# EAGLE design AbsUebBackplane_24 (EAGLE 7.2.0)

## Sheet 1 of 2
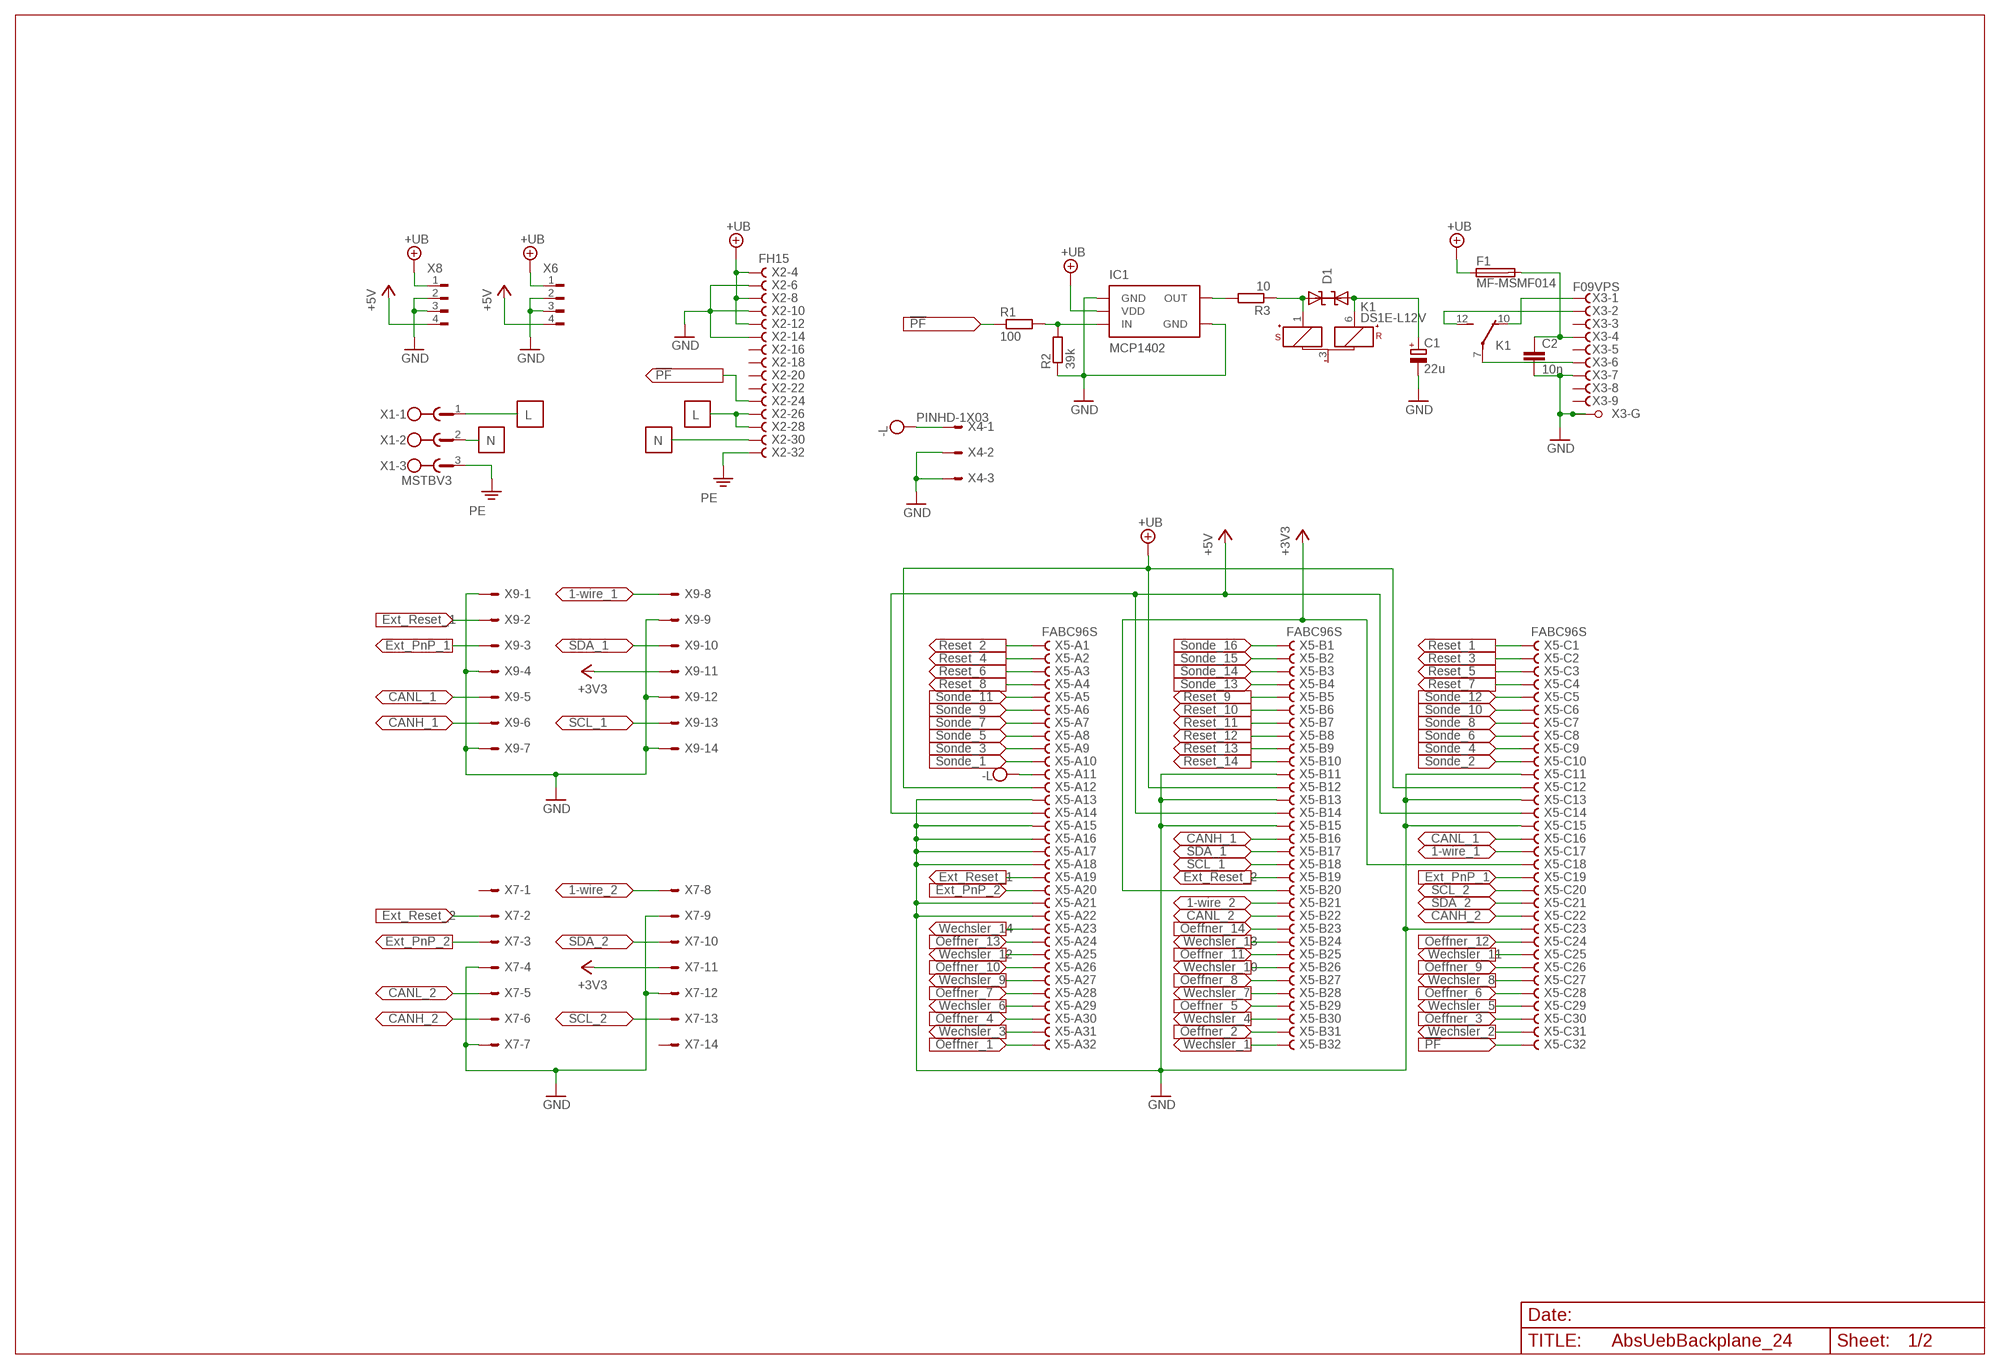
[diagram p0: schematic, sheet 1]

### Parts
C1  22u  CPOL-2-5  [RAD-FR-2,0-5]
C2  10n  C-SMD-1206  [C1206]
D1  P6SMB11CAT3  [SMB-DO-214AA]
F1  MF-MSMF014  [MF-MSMF-S1]
IC1  MCP1402  [SOT223-5]
K1  DS1E-L12V  [DS1E-L]
R1  100  R-SMD-1206  [R1206]
R2  39k  R-SMD-1206  [R1206]
R3  10  R-SMD-1206  [R1206]
X1  MSTBV3  [MSTBV3]
X2  FH15  [FH15]
X3  F09VPS  [F09VP]
X4  PINHD-1X03  [PINHD-1X03_LOCK]
X5  FABC96S  [FABC96S]
X6  FLOPPY-4  [FLOPPY-4]
X7  ML14E  [ML14]
X8  FLOPPY-4  [FLOPPY-4]
X9  ML14E  [ML14]

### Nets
1-WIRE_1: X5.C17 X9.8
1-WIRE_2: X5.B21 X7.8
!PF: R1.1 X2.24 X5.C32
+3V3: X5.B20 X5.C18 X7.11 X9.11
+5V: X5.A14 X5.B14 X5.C14 X6.4 X8.4
+UB: F1.1 IC1.2(VDD) X2.4 X2.8 X2.12 X5.A12 X5.B12 X5.C12 X6.1 X8.1 ; also sheet 2
-L: X4.1 X5.A11 ; also sheet 2
CANH_1: X5.B16 X9.6
CANH_2: X5.C22 X7.6
CANL_1: X5.C16 X9.5
CANL_2: X5.B22 X7.5
EXT_PNP_1: X5.C19 X9.3
EXT_PNP_2: X5.A20 X7.3
EXT_RESET_1: X5.A19 X9.2
EXT_RESET_2: X5.B19 X7.2
GND: C1.- C2.2 IC1.1(GND) IC1.4(GND) R2.1 X2.6 X2.10 X2.14 X3.7(-7:F) X3.G1(-G:G1) X3.G2(-G:G2) X4.2 X4.3 X5.A13 X5.A15 X5.A16 X5.A17 X5.A18 X5.A21 X5.A22 X5.B11 X5.B13 X5.B15 X5.C11 X5.C13 X5.C15 X5.C23 X6.2 X6.3 X7.4 X7.7 X7.9 X7.12 X8.2 X8.3 X9.1 X9.4 X9.7 X9.9 X9.12 X9.14 ; also sheet 2
L: X1.1 X2.26 X2.28
N: X1.2 X2.30
N$1: D1.1(C) K1.1(1:S+) R3.1
N$2: IC1.3(IN) R1.2 R2.2
N$3: C1.+ D1.2(A) K1.6(1:R+)
N$4: IC1.5(OUT) R3.2
N$5: K1.7(2:P) X3.6(-6:F)
N$6: K1.10(2:O) X3.1(-1:F)
N$7: K1.12(2:S) X3.2(-2:F)
N$8: C2.1 F1.2 X3.4(-4:F)
OEFFNER_1: X5.A32 ; also sheet 2
OEFFNER_2: X5.B31 ; also sheet 2
OEFFNER_3: X5.C30 ; also sheet 2
OEFFNER_4: X5.A30 ; also sheet 2
OEFFNER_5: X5.B29 ; also sheet 2
OEFFNER_6: X5.C28 ; also sheet 2
OEFFNER_7: X5.A28 ; also sheet 2
OEFFNER_8: X5.B27 ; also sheet 2
OEFFNER_9: X5.C26 ; also sheet 2
OEFFNER_10: X5.A26 ; also sheet 2
OEFFNER_11: X5.B25 ; also sheet 2
OEFFNER_12: X5.C24 ; also sheet 2
OEFFNER_13: X5.A24 ; also sheet 2
OEFFNER_14: X5.B23 ; also sheet 2
PE: X1.3 X2.32
RESET_1: X5.C1 ; also sheet 2
RESET_2: X5.A1 ; also sheet 2
RESET_3: X5.C2 ; also sheet 2
RESET_4: X5.A2 ; also sheet 2
RESET_5: X5.C3 ; also sheet 2
RESET_6: X5.A3 ; also sheet 2
RESET_7: X5.C4 ; also sheet 2
RESET_8: X5.A4 ; also sheet 2
RESET_9: X5.B5 ; also sheet 2
RESET_10: X5.B6 ; also sheet 2
RESET_11: X5.B7 ; also sheet 2
RESET_12: X5.B8 ; also sheet 2
RESET_13: X5.B9 ; also sheet 2
RESET_14: X5.B10 ; also sheet 2
SCL_1: X5.B18 X9.13
SCL_2: X5.C20 X7.13
SDA_1: X5.B17 X9.10
SDA_2: X5.C21 X7.10
SONDE_1: X5.A10 ; also sheet 2
SONDE_2: X5.C10 ; also sheet 2
SONDE_3: X5.A9 ; also sheet 2
SONDE_4: X5.C9 ; also sheet 2
SONDE_5: X5.A8 ; also sheet 2
SONDE_6: X5.C8 ; also sheet 2
SONDE_7: X5.A7 ; also sheet 2
SONDE_8: X5.C7 ; also sheet 2
SONDE_9: X5.A6 ; also sheet 2
SONDE_10: X5.C6 ; also sheet 2
SONDE_11: X5.A5 ; also sheet 2
SONDE_12: X5.C5 ; also sheet 2
SONDE_13: X5.B4 ; also sheet 2
SONDE_14: X5.B3 ; also sheet 2
SONDE_15: X5.B2
SONDE_16: X5.B1
WECHSLER_1: X5.B32 ; also sheet 2
WECHSLER_2: X5.C31 ; also sheet 2
WECHSLER_3: X5.A31 ; also sheet 2
WECHSLER_4: X5.B30 ; also sheet 2
WECHSLER_5: X5.C29 ; also sheet 2
WECHSLER_6: X5.A29 ; also sheet 2
WECHSLER_7: X5.B28 ; also sheet 2
WECHSLER_8: X5.C27 ; also sheet 2
WECHSLER_9: X5.A27 ; also sheet 2
WECHSLER_10: X5.B26 ; also sheet 2
WECHSLER_11: X5.C25 ; also sheet 2
WECHSLER_12: X5.A25 ; also sheet 2
WECHSLER_13: X5.B24 ; also sheet 2
WECHSLER_14: X5.A23 ; also sheet 2
Unconnected: K1.3(1:-) X2.16 X2.18 X2.20 X2.22 X3.3(-3:F) X3.5(-5:F) X3.8(-8:F) X3.9(-9:F) X7.1 X7.14

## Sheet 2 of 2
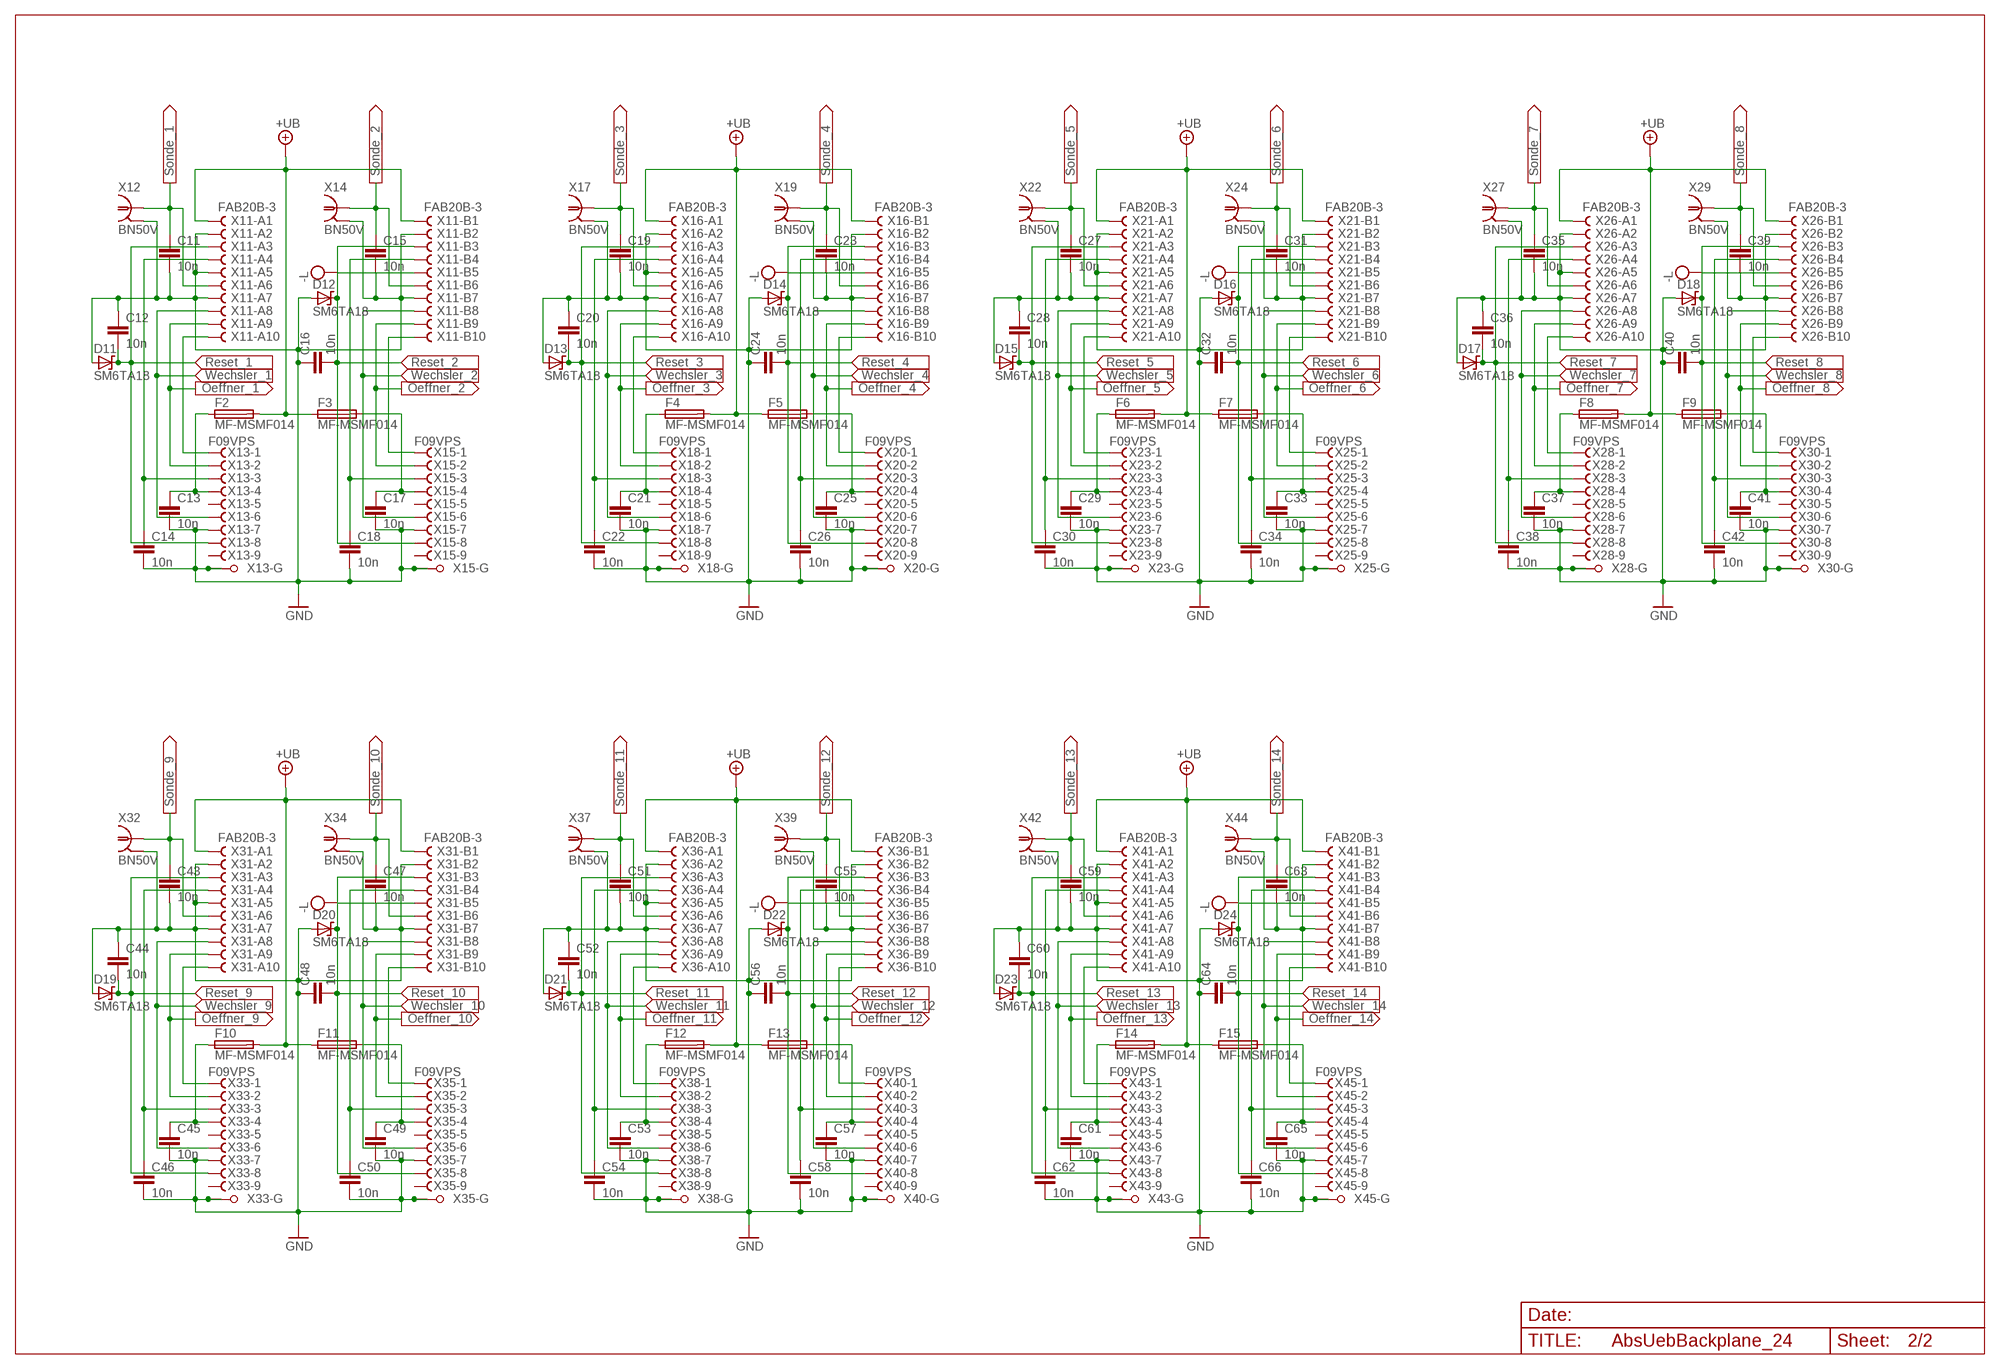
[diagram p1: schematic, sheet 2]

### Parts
C11  10n  C-SMD-1206  [C1206]
C12  10n  C-SMD-1206  [C1206]
C13  10n  C-SMD-1206  [C1206]
C14  10n  C-SMD-1206  [C1206]
C15  10n  C-SMD-1206  [C1206]
C16  10n  C-SMD-1206  [C1206]
C17  10n  C-SMD-1206  [C1206]
C18  10n  C-SMD-1206  [C1206]
C19  10n  C-SMD-1206  [C1206]
C20  10n  C-SMD-1206  [C1206]
C21  10n  C-SMD-1206  [C1206]
C22  10n  C-SMD-1206  [C1206]
C23  10n  C-SMD-1206  [C1206]
C24  10n  C-SMD-1206  [C1206]
C25  10n  C-SMD-1206  [C1206]
C26  10n  C-SMD-1206  [C1206]
C27  10n  C-SMD-1206  [C1206]
C28  10n  C-SMD-1206  [C1206]
C29  10n  C-SMD-1206  [C1206]
C30  10n  C-SMD-1206  [C1206]
C31  10n  C-SMD-1206  [C1206]
C32  10n  C-SMD-1206  [C1206]
C33  10n  C-SMD-1206  [C1206]
C34  10n  C-SMD-1206  [C1206]
C35  10n  C-SMD-1206  [C1206]
C36  10n  C-SMD-1206  [C1206]
C37  10n  C-SMD-1206  [C1206]
C38  10n  C-SMD-1206  [C1206]
C39  10n  C-SMD-1206  [C1206]
C40  10n  C-SMD-1206  [C1206]
C41  10n  C-SMD-1206  [C1206]
C42  10n  C-SMD-1206  [C1206]
C43  10n  C-SMD-1206  [C1206]
C44  10n  C-SMD-1206  [C1206]
C45  10n  C-SMD-1206  [C1206]
C46  10n  C-SMD-1206  [C1206]
C47  10n  C-SMD-1206  [C1206]
C48  10n  C-SMD-1206  [C1206]
C49  10n  C-SMD-1206  [C1206]
C50  10n  C-SMD-1206  [C1206]
C51  10n  C-SMD-1206  [C1206]
C52  10n  C-SMD-1206  [C1206]
C53  10n  C-SMD-1206  [C1206]
C54  10n  C-SMD-1206  [C1206]
C55  10n  C-SMD-1206  [C1206]
C56  10n  C-SMD-1206  [C1206]
C57  10n  C-SMD-1206  [C1206]
C58  10n  C-SMD-1206  [C1206]
C59  10n  C-SMD-1206  [C1206]
C60  10n  C-SMD-1206  [C1206]
C61  10n  C-SMD-1206  [C1206]
C62  10n  C-SMD-1206  [C1206]
C63  10n  C-SMD-1206  [C1206]
C64  10n  C-SMD-1206  [C1206]
C65  10n  C-SMD-1206  [C1206]
C66  10n  C-SMD-1206  [C1206]
D11  SM6TA18  [DO-214AA]
D12  SM6TA18  [DO-214AA]
D13  SM6TA18  [DO-214AA]
D14  SM6TA18  [DO-214AA]
D15  SM6TA18  [DO-214AA]
D16  SM6TA18  [DO-214AA]
D17  SM6TA18  [DO-214AA]
D18  SM6TA18  [DO-214AA]
D19  SM6TA18  [DO-214AA]
D20  SM6TA18  [DO-214AA]
D21  SM6TA18  [DO-214AA]
D22  SM6TA18  [DO-214AA]
D23  SM6TA18  [DO-214AA]
D24  SM6TA18  [DO-214AA]
F2  MF-MSMF014  [MF-MSMF-S1]
F3  MF-MSMF014  [MF-MSMF-S1]
F4  MF-MSMF014  [MF-MSMF-S1]
F5  MF-MSMF014  [MF-MSMF-S1]
F6  MF-MSMF014  [MF-MSMF-S1]
F7  MF-MSMF014  [MF-MSMF-S1]
F8  MF-MSMF014  [MF-MSMF-S1]
F9  MF-MSMF014  [MF-MSMF-S1]
F10  MF-MSMF014  [MF-MSMF-S1]
F11  MF-MSMF014  [MF-MSMF-S1]
F12  MF-MSMF014  [MF-MSMF-S1]
F13  MF-MSMF014  [MF-MSMF-S1]
F14  MF-MSMF014  [MF-MSMF-S1]
F15  MF-MSMF014  [MF-MSMF-S1]
X11  FAB20B-3  [FAB20B-3]
X12  BN50V  [BN50V]
X13  F09VPS  [F09VP]
X14  BN50V  [BN50V]
X15  F09VPS  [F09VP]
X16  FAB20B-3  [FAB20B-3]
X17  BN50V  [BN50V]
X18  F09VPS  [F09VP]
X19  BN50V  [BN50V]
X20  F09VPS  [F09VP]
X21  FAB20B-3  [FAB20B-3]
X22  BN50V  [BN50V]
X23  F09VPS  [F09VP]
X24  BN50V  [BN50V]
X25  F09VPS  [F09VP]
X26  FAB20B-3  [FAB20B-3]
X27  BN50V  [BN50V]
X28  F09VPS  [F09VP]
X29  BN50V  [BN50V]
X30  F09VPS  [F09VP]
X31  FAB20B-3  [FAB20B-3]
X32  BN50V  [BN50V]
X33  F09VPS  [F09VP]
X34  BN50V  [BN50V]
X35  F09VPS  [F09VP]
X36  FAB20B-3  [FAB20B-3]
X37  BN50V  [BN50V]
X38  F09VPS  [F09VP]
X39  BN50V  [BN50V]
X40  F09VPS  [F09VP]
X41  FAB20B-3  [FAB20B-3]
X42  BN50V  [BN50V]
X43  F09VPS  [F09VP]
X44  BN50V  [BN50V]
X45  F09VPS  [F09VP]

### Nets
+UB: F2.2 F3.1 F4.2 F5.1 F6.2 F7.1 F8.2 F9.1 F10.2 F11.1 F12.2 F13.1 F14.2 F15.1 X11.A1 X11.B1 X16.A1 X16.B1 X21.A1 X21.B1 X26.A1 X26.B1 X31.A1 X31.B1 X36.A1 X36.B1 X41.A1 X41.B1 ; also sheet 1
-L: X11.B5 X16.B5 X21.B5 X26.B5 X31.B5 X36.B5 X41.B5 ; also sheet 1
GND: C11.2 C12.1 C13.2 C14.2 C15.2 C16.1 C17.2 C18.2 C19.2 C20.1 C21.2 C22.2 C23.2 C24.1 C25.2 C26.2 C27.2 C28.1 C29.2 C30.2 C31.2 C32.1 C33.2 C34.2 C35.2 C36.1 C37.2 C38.2 C39.2 C40.1 C41.2 C42.2 C43.2 C44.1 C45.2 C46.2 C47.2 C48.1 C49.2 C50.2 C51.2 C52.1 C53.2 C54.2 C55.2 C56.1 C57.2 C58.2 C59.2 C60.1 C61.2 C62.2 C63.2 C64.1 C65.2 C66.2 D11.1(A) D12.1(A) D13.1(A) D14.1(A) D15.1(A) D16.1(A) D17.1(A) D18.1(A) D19.1(A) D20.1(A) D21.1(A) D22.1(A) D23.1(A) D24.1(A) X11.A2 X11.A5 X11.A7 X11.B2 X11.B7 X12.2 X12.3 X12.4 X12.5 X13.7(-7:F) X13.G1(-G:G1) X13.G2(-G:G2) X14.2 X14.3 X14.4 X14.5 X15.7(-7:F) X15.G1(-G:G1) X15.G2(-G:G2) X16.A2 X16.A5 X16.A7 X16.B2 X16.B7 X17.2 X17.3 X17.4 X17.5 X18.7(-7:F) X18.G1(-G:G1) X18.G2(-G:G2) X19.2 X19.3 X19.4 X19.5 X20.7(-7:F) X20.G1(-G:G1) X20.G2(-G:G2) X21.A2 X21.A5 X21.A7 X21.B2 X21.B7 X22.2 X22.3 X22.4 X22.5 X23.7(-7:F) X23.G1(-G:G1) X23.G2(-G:G2) X24.2 X24.3 X24.4 X24.5 X25.7(-7:F) X25.G1(-G:G1) X25.G2(-G:G2) X26.A2 X26.A5 X26.A7 X26.B2 X26.B7 X27.2 X27.3 X27.4 X27.5 X28.7(-7:F) X28.G1(-G:G1) X28.G2(-G:G2) X29.2 X29.3 X29.4 X29.5 X30.7(-7:F) X30.G1(-G:G1) X30.G2(-G:G2) X31.A2 X31.A5 X31.A7 X31.B2 X31.B7 X32.2 X32.3 X32.4 X32.5 X33.7(-7:F) X33.G1(-G:G1) X33.G2(-G:G2) X34.2 X34.3 X34.4 X34.5 X35.7(-7:F) X35.G1(-G:G1) X35.G2(-G:G2) X36.A2 X36.A5 X36.A7 X36.B2 X36.B7 X37.2 X37.3 X37.4 X37.5 X38.7(-7:F) X38.G1(-G:G1) X38.G2(-G:G2) X39.2 X39.3 X39.4 X39.5 X40.7(-7:F) X40.G1(-G:G1) X40.G2(-G:G2) X41.A2 X41.A5 X41.A7 X41.B2 X41.B7 X42.2 X42.3 X42.4 X42.5 X43.7(-7:F) X43.G1(-G:G1) X43.G2(-G:G2) X44.2 X44.3 X44.4 X44.5 X45.7(-7:F) X45.G1(-G:G1) X45.G2(-G:G2) ; also sheet 1
MESSSIG_1: C14.1 X11.A4 X13.3(-3:F)
MESSSIG_2: C18.1 X11.B4 X15.3(-3:F)
MESSSIG_3: C22.1 X16.A4 X18.3(-3:F)
MESSSIG_4: C26.1 X16.B4 X20.3(-3:F)
MESSSIG_5: C30.1 X21.A4 X23.3(-3:F)
MESSSIG_6: C34.1 X21.B4 X25.3(-3:F)
MESSSIG_7: C38.1 X26.A4 X28.3(-3:F)
MESSSIG_8: C42.1 X26.B4 X30.3(-3:F)
MESSSIG_9: C46.1 X31.A4 X33.3(-3:F)
MESSSIG_10: C50.1 X31.B4 X35.3(-3:F)
MESSSIG_11: C54.1 X36.A4 X38.3(-3:F)
MESSSIG_12: C58.1 X36.B4 X40.3(-3:F)
MESSSIG_13: C62.1 X41.A4 X43.3(-3:F)
MESSSIG_14: C66.1 X41.B4 X45.3(-3:F)
N$9: C13.1 F2.1 X13.4(-4:F)
N$10: C17.1 F3.2 X15.4(-4:F)
N$11: C21.1 F4.1 X18.4(-4:F)
N$12: C37.1 F8.1 X28.4(-4:F)
N$21: C29.1 F6.1 X23.4(-4:F)
N$22: C45.1 F10.1 X33.4(-4:F)
N$23: C53.1 F12.1 X38.4(-4:F)
N$24: C61.1 F14.1 X43.4(-4:F)
N$25: C25.1 F5.2 X20.4(-4:F)
N$26: C33.1 F7.2 X25.4(-4:F)
N$27: C41.1 F9.2 X30.4(-4:F)
N$28: C65.1 F15.2 X45.4(-4:F)
N$29: C57.1 F13.2 X40.4(-4:F)
N$30: C49.1 F11.2 X35.4(-4:F)
OEFFNER_1: X11.A9 X13.2(-2:F) ; also sheet 1
OEFFNER_2: X11.B9 X15.2(-2:F) ; also sheet 1
OEFFNER_3: X16.A9 X18.2(-2:F) ; also sheet 1
OEFFNER_4: X16.B9 X20.2(-2:F) ; also sheet 1
OEFFNER_5: X21.A9 X23.2(-2:F) ; also sheet 1
OEFFNER_6: X21.B9 X25.2(-2:F) ; also sheet 1
OEFFNER_7: X26.A9 X28.2(-2:F) ; also sheet 1
OEFFNER_8: X26.B9 X30.2(-2:F) ; also sheet 1
OEFFNER_9: X31.A9 X33.2(-2:F) ; also sheet 1
OEFFNER_10: X31.B9 X35.2(-2:F) ; also sheet 1
OEFFNER_11: X36.A9 X38.2(-2:F) ; also sheet 1
OEFFNER_12: X36.B9 X40.2(-2:F) ; also sheet 1
OEFFNER_13: X41.A9 X43.2(-2:F) ; also sheet 1
OEFFNER_14: X41.B9 X45.2(-2:F) ; also sheet 1
RESET_1: C12.2 D11.2(C) X11.A3 X13.8(-8:F) ; also sheet 1
RESET_2: C16.2 D12.2(C) X11.B3 X15.8(-8:F) ; also sheet 1
RESET_3: C20.2 D13.2(C) X16.A3 X18.8(-8:F) ; also sheet 1
RESET_4: C24.2 D14.2(C) X16.B3 X20.8(-8:F) ; also sheet 1
RESET_5: C28.2 D15.2(C) X21.A3 X23.8(-8:F) ; also sheet 1
RESET_6: C32.2 D16.2(C) X21.B3 X25.8(-8:F) ; also sheet 1
RESET_7: C36.2 D17.2(C) X26.A3 X28.8(-8:F) ; also sheet 1
RESET_8: C40.2 D18.2(C) X26.B3 X30.8(-8:F) ; also sheet 1
RESET_9: C44.2 D19.2(C) X31.A3 X33.8(-8:F) ; also sheet 1
RESET_10: C48.2 D20.2(C) X31.B3 X35.8(-8:F) ; also sheet 1
RESET_11: C52.2 D21.2(C) X36.A3 X38.8(-8:F) ; also sheet 1
RESET_12: C56.2 D22.2(C) X36.B3 X40.8(-8:F) ; also sheet 1
RESET_13: C60.2 D23.2(C) X41.A3 X43.8(-8:F) ; also sheet 1
RESET_14: C64.2 D24.2(C) X41.B3 X45.8(-8:F) ; also sheet 1
SCHLIESSER_1: X11.A10 X13.1(-1:F)
SCHLIESSER_2: X11.B10 X15.1(-1:F)
SCHLIESSER_3: X16.A10 X18.1(-1:F)
SCHLIESSER_4: X16.B10 X20.1(-1:F)
SCHLIESSER_5: X21.A10 X23.1(-1:F)
SCHLIESSER_6: X21.B10 X25.1(-1:F)
SCHLIESSER_7: X26.A10 X28.1(-1:F)
SCHLIESSER_8: X26.B10 X30.1(-1:F)
SCHLIESSER_9: X31.A10 X33.1(-1:F)
SCHLIESSER_10: X31.B10 X35.1(-1:F)
SCHLIESSER_11: X36.A10 X38.1(-1:F)
SCHLIESSER_12: X36.B10 X40.1(-1:F)
SCHLIESSER_13: X41.A10 X43.1(-1:F)
SCHLIESSER_14: X41.B10 X45.1(-1:F)
SONDE_1: C11.1 X11.A6 X12.1 ; also sheet 1
SONDE_2: C15.1 X11.B6 X14.1 ; also sheet 1
SONDE_3: C19.1 X16.A6 X17.1 ; also sheet 1
SONDE_4: C23.1 X16.B6 X19.1 ; also sheet 1
SONDE_5: C27.1 X21.A6 X22.1 ; also sheet 1
SONDE_6: C31.1 X21.B6 X24.1 ; also sheet 1
SONDE_7: C35.1 X26.A6 X27.1 ; also sheet 1
SONDE_8: C39.1 X26.B6 X29.1 ; also sheet 1
SONDE_9: C43.1 X31.A6 X32.1 ; also sheet 1
SONDE_10: C47.1 X31.B6 X34.1 ; also sheet 1
SONDE_11: C51.1 X36.A6 X37.1 ; also sheet 1
SONDE_12: C55.1 X36.B6 X39.1 ; also sheet 1
SONDE_13: C59.1 X41.A6 X42.1 ; also sheet 1
SONDE_14: C63.1 X41.B6 X44.1 ; also sheet 1
WECHSLER_1: X11.A8 X13.6(-6:F) ; also sheet 1
WECHSLER_2: X11.B8 X15.6(-6:F) ; also sheet 1
WECHSLER_3: X16.A8 X18.6(-6:F) ; also sheet 1
WECHSLER_4: X16.B8 X20.6(-6:F) ; also sheet 1
WECHSLER_5: X21.A8 X23.6(-6:F) ; also sheet 1
WECHSLER_6: X21.B8 X25.6(-6:F) ; also sheet 1
WECHSLER_7: X26.A8 X28.6(-6:F) ; also sheet 1
WECHSLER_8: X26.B8 X30.6(-6:F) ; also sheet 1
WECHSLER_9: X31.A8 X33.6(-6:F) ; also sheet 1
WECHSLER_10: X31.B8 X35.6(-6:F) ; also sheet 1
WECHSLER_11: X36.A8 X38.6(-6:F) ; also sheet 1
WECHSLER_12: X36.B8 X40.6(-6:F) ; also sheet 1
WECHSLER_13: X41.A8 X43.6(-6:F) ; also sheet 1
WECHSLER_14: X41.B8 X45.6(-6:F) ; also sheet 1
Unconnected: X13.5(-5:F) X13.9(-9:F) X15.5(-5:F) X15.9(-9:F) X18.5(-5:F) X18.9(-9:F) X20.5(-5:F) X20.9(-9:F) X23.5(-5:F) X23.9(-9:F) X25.5(-5:F) X25.9(-9:F) X28.5(-5:F) X28.9(-9:F) X30.5(-5:F) X30.9(-9:F) X33.5(-5:F) X33.9(-9:F) X35.5(-5:F) X35.9(-9:F) X38.5(-5:F) X38.9(-9:F) X40.5(-5:F) X40.9(-9:F) X43.5(-5:F) X43.9(-9:F) X45.5(-5:F) X45.9(-9:F)

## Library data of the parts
C1 = AbsUebParts_11:CPOL-2-5: Elektrolytkondensator RM 2,0mm; MF: Panasonic; OC_REICHELT: RAD FR 22/50
C2 C11-C66 = AbsUebParts_11:C-SMD: SMD Keramik Vielschichtkondensatoren
D1 = AbsUebParts_11:P6SMB11CAT3: Suppressor diode bi-directional
D11-D24 = AbsUebParts_11:SM6TA: STM Transil Suppressor Diode; MF: STM; MPN: SM6T18A; OC_REICHELT: P6SMB 18A SMD
F1-F15 = AbsUebParts_11:MF-MSMF: Bourns MF-MSMF Series; MF: Bourns; MPN: MF-MSMF014-2; OC_RS: 647-8162
IC1 = AbsUebParts_11:MCP1402: MCP1402 500mA. High-Speed Power MOSFET Driver; MF: Microchip; MPN: MCP1402; OC_RS: 668-4203
K1 = AbsUebParts_11:DS1E-L*: DS-RELAYS HIGHLY SENSITIVE 1500 V FCC SURGE NAiS WITHSTANDING MINIATURE RELAY Source: http://www.mew-europe.com/.. en_ds_61005_0001.pdf; MF: Panasonic; MPN: DS2E-SL2-DC12V; OC_RS: 815-4988
R1-R3 = AbsUebParts_11:R-SMD: SMD Resistor
X1 = AbsUebParts_11:MSTBV3: FCI Anschlussleiste, 3 pins, 5.08mm; MF: FCI; MPN: 20020107-H031A01LF; OC_RS: 707-5424
X2 = AbsUebParts_11:FH15: CONNECTOR female, 15 pins, type H, rows DZ; OC_REICHELT: FL-H 15G
X3 X13 X15 X18 X20 X23 X25 X28 X30 X33 X35 X38 X40 X43 X45 = AbsUebParts_11:F09VPS: 9 pins female SUB-D Amphenol, female, 9 pins, vertical, standoff boardlock; MF: AMP; MPN: L77SD EH09S OL2 RM5; OC_RS: 615-6171
X4 = AbsUebParts_11:PINHD-1X03: PINHEADER 1X3 RM 2.54 mm; OC_REICHELT: MPE 087-1-003
X5 = AbsUebParts_11:FABC96S: CONNECTOR female, 96 pins, type R, rows ABC, grid 2.54 mm; MF: ept; OC_REICHELT: FL-C 96G4
X6 X8 = AbsUebParts_11:FLOPPY-4: MATE N-LOCK Floppy / HDD conector, 4 pins, 250V, 6A; OC_REICHELT: PSG 5
X7 X9 = AbsUebParts_11:ML14E: HARTING; OC_REICHELT: PSL 14
X11 X16 X21 X26 X31 X36 X41 = AbsUebParts_11:FAB20B-3: CONNECTOR female, 20 pins, type B/3, rows AB, grid 2.54 mm; OC_REICHELT: FL-B3 20G; OC_RS: 693-1919
X12 X14 X17 X19 X22 X24 X27 X29 X32 X34 X37 X39 X42 X44 = AbsUebParts_11:BN50V: BNC CONNECTOR VERTICAL; MF: TE; MPN: 5413969-2; OC_RS: 710-0214

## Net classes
0 default: clearance 0.205 mm

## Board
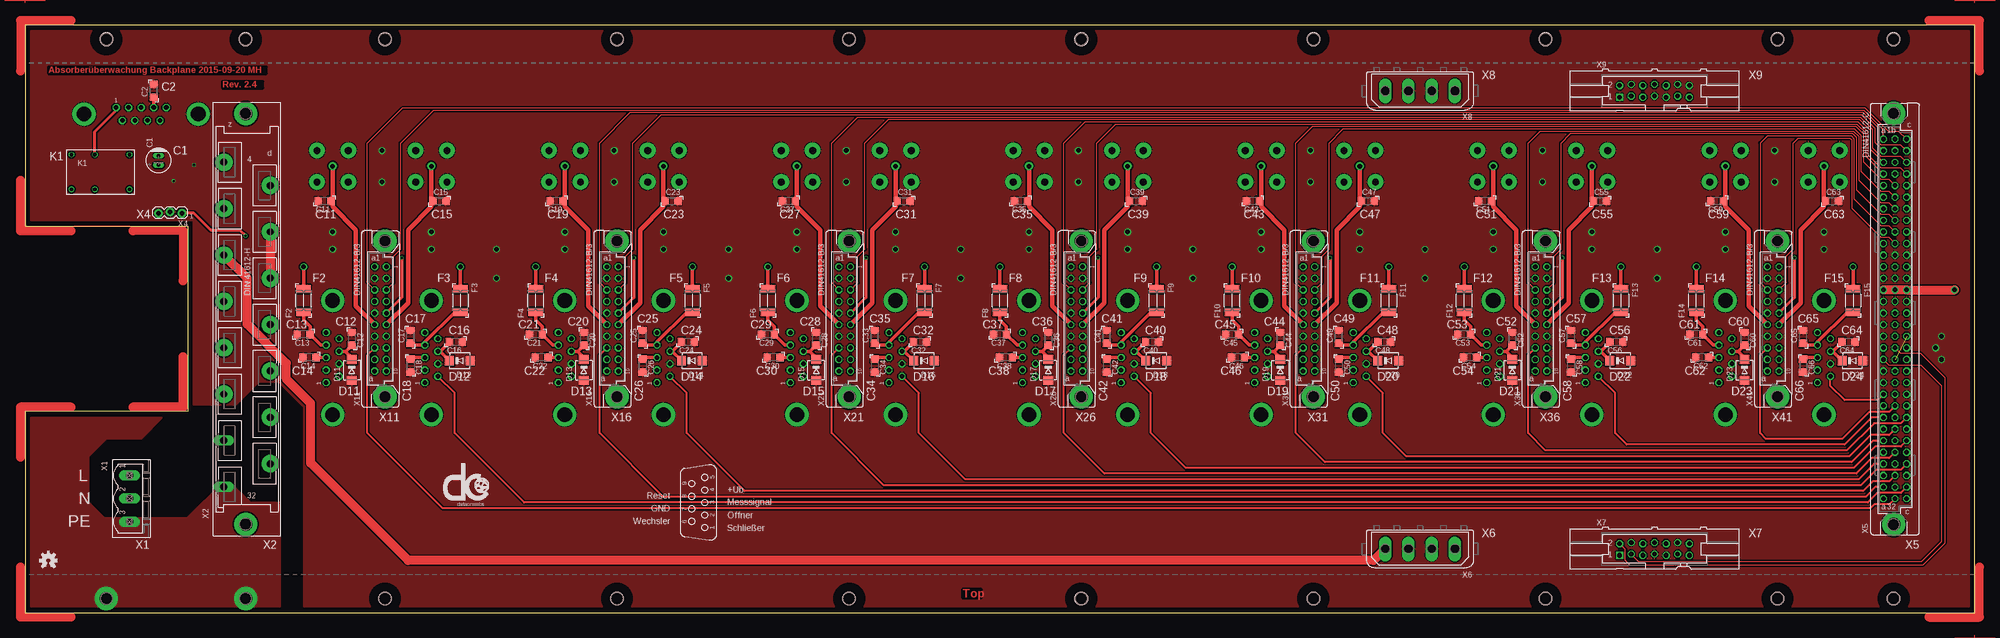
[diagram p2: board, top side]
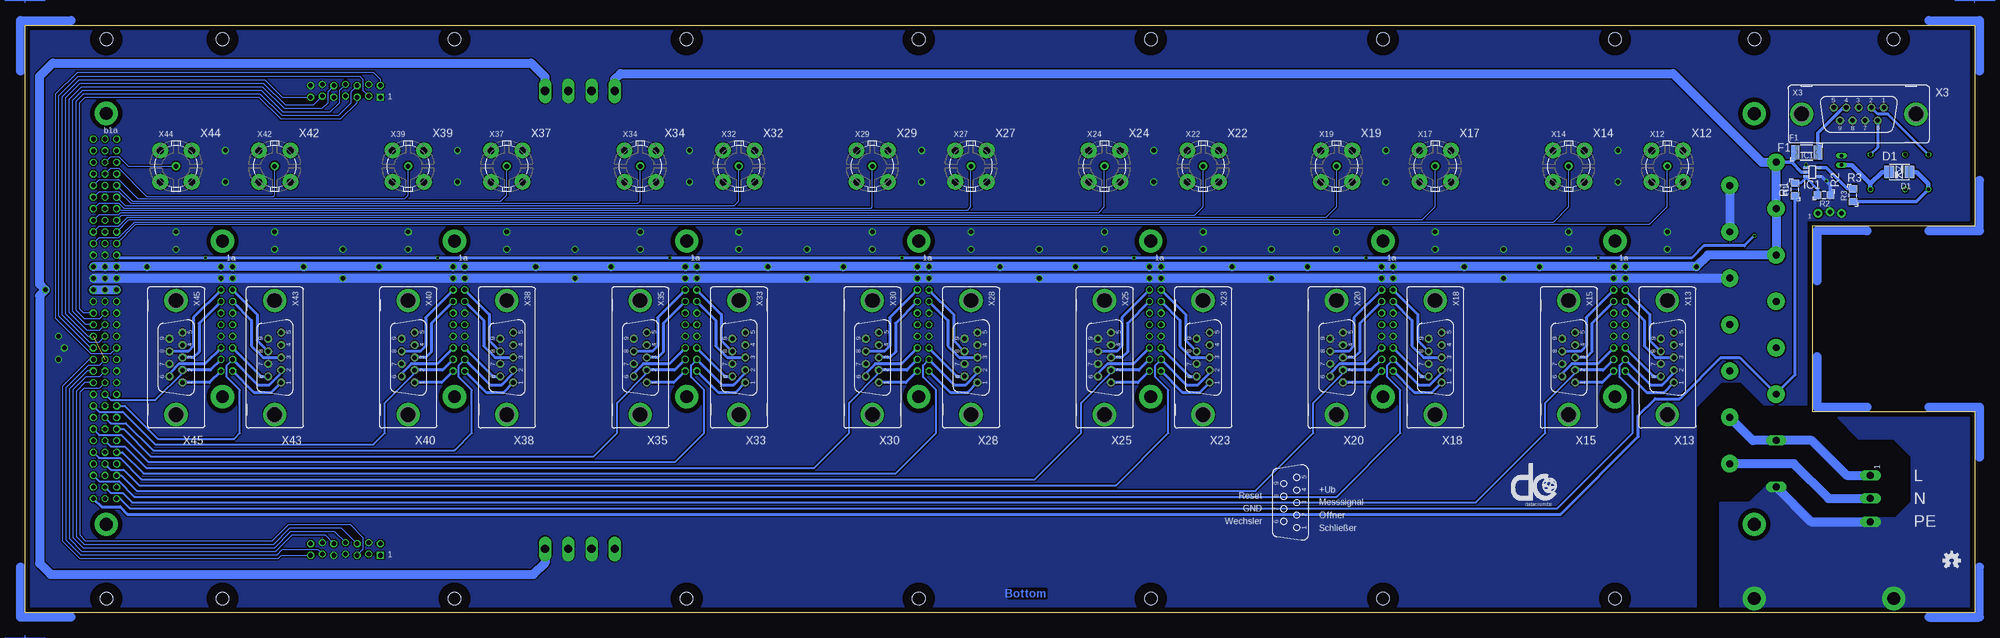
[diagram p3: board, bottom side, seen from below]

Size 426.72 x 128.7 mm. Coordinates in mm from the lower left corner, seen from the top.
Outline: 0,0 426.72,0 426.72,128.7 0,128.7 0,84.67 35.56,84.67 35.56,44.03 0,44.03 0,0
Copper layers (1*16): Top 0.018mm / dielectric 1.55mm / Bottom 0.018mm
Design rules "eC_2Layer_PClass6_BaseCopperO18_eCDefault *": minimum track width 0.15mm, minimum drill 0.35mm, track to track 0.15mm, track to pad 0.15mm, pad to pad 0.15mm, via to via 0.15mm, smd to smd 0mil, copper to edge 0.25mm, drill to drill 0.35mm, minimum pad ring 0.175mm, minimum via ring 0.125mm, stop-mask expansion 0mil, vias tented up to drill 20mil, thermal gap 0.2mm
Holes 2.8 mm at 48.26,125.6 78.74,125.6 129.54,125.6 180.34,125.6 231.14,125.6 281.94,125.6 332.74,125.6 383.54,125.6 78.74,3.1 129.54,3.1 180.34,3.1 231.14,3.1 281.94,3.1 332.74,3.1 383.54,3.1 17.78,125.6 408.94,125.6 408.94,3.1
tRestrict: area 76.5,0.8 to 81,5.4; area 127.3,0.8 to 131.8,5.4; area 178.1,0.8 to 182.6,5.4; area 228.9,0.8 to 233.4,5.4; area 279.7,0.8 to 284.2,5.4; area 330.5,0.8 to 335,5.4; area 381.3,0.8 to 385.8,5.4; area 406.7,0.8 to 411.2,5.4; area 381.3,123.3 to 385.8,127.9; area 406.7,123.3 to 411.2,127.9; area 330.5,123.3 to 335,127.9; area 279.7,123.3 to 284.2,127.9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
bRestrict: area 76.5,0.8 to 81,5.4; area 127.3,0.8 to 131.8,5.4; area 178.1,0.8 to 182.6,5.4; area 228.9,0.8 to 233.4,5.4; area 279.7,0.8 to 284.2,5.4; area 330.5,0.8 to 335,5.4; area 381.3,0.8 to 385.8,5.4; area 406.7,0.8 to 411.2,5.4; area 381.3,123.3 to 385.8,127.9; area 406.7,123.3 to 411.2,127.9; area 330.5,123.3 to 335,127.9; area 279.7,123.3 to 284.2,127.9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
vRestrict: area 330.5,0.8 to 335,5.4; area 381.3,0.8 to 385.8,5.4; area 406.7,0.8 to 411.2,5.4; area 279.7,0.8 to 284.2,5.4; area 228.9,0.8 to 233.4,5.4; area 178.1,0.8 to 182.6,5.4; area 127.3,0.8 to 131.8,5.4; area 76.5,0.8 to 81,5.4; area 46,0.8 to 50.5,5.4; area 15.5,0.8 to 20.1,5.4; area 15.5,123.3 to 20.1,127.9; area 46,123.3 to 50.5,127.9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

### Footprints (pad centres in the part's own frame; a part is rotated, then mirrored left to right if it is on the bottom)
RAD-FR-2,0-5 = drill 0.8 long: + -1,0; - 1,0
C1206 = smd 1.6 x 1.8: 1 -1.4,0; 2 1.4,0
SMB-DO-214AA = smd 2.16 x 2.75: 1 -2.2,0; 2 2.2,0
DO-214AA = smd 1.96 x 2.18: 1 -2.28,0; 2 2.28,0
MF-MSMF-S1 = smd 1.78 x 3.2: 1 -2.49,0; 2 2.49,0
SOT223-5 = smd 0.6 x 1.1: 1 -0.95,-1.4; 2 0,-1.4; 3 0.95,-1.4; 4 0.95,1.4; 5 -0.95,1.4
DS1E-L = drill 0.8: 1 -6.35,-3.81; 3 -1.27,-3.81; 6 6.35,-3.81; 7 6.35,3.81; 10 -1.27,3.81; 12 -6.35,3.81
R1206 = smd 1.6 x 1.8: 1 -1.4,0; 2 1.4,0
MSTBV3 = drill 1.5 pad 2.184 long: 1 -5.08,0; 2 0,0; 3 5.08,0
FH15 = drill 1.5 pad 3.81: 4 -5.08,34.315; 6 5.08,29.235; 8 -5.08,24.155; 10 5.08,19.075; 12 -5.08,13.995; 14 5.08,8.915; 16 -5.08,3.835; 18 5.08,-1.245; 20 -5.08,-6.325; 22 5.08,-11.405; 24 -5.08,-16.485; 26 5.08,-21.565; 30 5.08,-31.725 | drill 1.5 pad 2.184 long: 28 -5.08,-26.645; 32 -5.08,-36.805 | drill 2.8 pad 5.08: X1 -0.305,44.983; X2 -0.305,-44.983
F09VP = drill 1 octagon: 1 5.486,1.422; 2 2.743,1.422; 3 0,1.422; 4 -2.743,1.422; 5 -5.486,1.422; 6 4.115,-1.422; 7 1.372,-1.422; 8 -1.372,-1.422; 9 -4.115,-1.422 | drill 3.2 pad 5.08: G1 -12.495,0; G2 12.495,0
PINHD-1X03_LOCK = drill 1 pad 1.88: 1 0,0.127; 2 2.54,-0.127; 3 5.08,0.127
FABC96S = drill 1 octagon: A1 -2.54,39.37; A2 -2.54,36.83; A3 -2.54,34.29; A4 -2.54,31.75; A5 -2.54,29.21; A6 -2.54,26.67; A7 -2.54,24.13; A8 -2.54,21.59; A9 -2.54,19.05; A10 -2.54,16.51; A11 -2.54,13.97; A12 -2.54,11.43; A13 -2.54,8.89; A14 -2.54,6.35; A15 -2.54,3.81; A16 -2.54,1.27; A17 -2.54,-1.27; A18 -2.54,-3.81; A19 -2.54,-6.35; A20 -2.54,-8.89; A21 -2.54,-11.43; A22 -2.54,-13.97; A23 -2.54,-16.51; A24 -2.54,-19.05; A25 -2.54,-21.59; A26 -2.54,-24.13; A27 -2.54,-26.67; A28 -2.54,-29.21; A29 -2.54,-31.75; A30 -2.54,-34.29; A31 -2.54,-36.83; A32 -2.54,-39.37; B1 0,39.37; B2 0,36.83; B3 0,34.29; B4 0,31.75; B5 0,29.21; B6 0,26.67; B7 0,24.13; B8 0,21.59; B9 0,19.05; B10 0,16.51; B11 0,13.97; B12 0,11.43; B13 0,8.89; B14 0,6.35; B15 0,3.81; B16 0,1.27; B17 0,-1.27; B18 0,-3.81; B19 0,-6.35; B20 0,-8.89; B21 0,-11.43; B22 0,-13.97; B23 0,-16.51; B24 0,-19.05; B25 0,-21.59; B26 0,-24.13; B27 0,-26.67; B28 0,-29.21; B29 0,-31.75; B30 0,-34.29; B31 0,-36.83; B32 0,-39.37; C1 2.54,39.37; C2 2.54,36.83; C3 2.54,34.29; C4 2.54,31.75; C5 2.54,29.21; C6 2.54,26.67; C7 2.54,24.13; C8 2.54,21.59; C9 2.54,19.05; C10 2.54,16.51; C11 2.54,13.97; C12 2.54,11.43; C13 2.54,8.89; C14 2.54,6.35; C15 2.54,3.81; C16 2.54,1.27; C17 2.54,-1.27; C18 2.54,-3.81; C19 2.54,-6.35; C20 2.54,-8.89; C21 2.54,-11.43; C22 2.54,-13.97; C23 2.54,-16.51; C24 2.54,-19.05; C25 2.54,-21.59; C26 2.54,-24.13; C27 2.54,-26.67; C28 2.54,-29.21; C29 2.54,-31.75; C30 2.54,-34.29; C31 2.54,-36.83; C32 2.54,-39.37 | drill 2.8 pad 5.08: X1 -0.305,45.009; X2 -0.305,-45.009
FLOPPY-4 = drill 1.8 pad 2.54 long: 1 7.62,0; 2 2.54,0; 3 -2.54,0; 4 -7.62,0
ML14 = drill 1 square: 1 -7.62,-1.397 | drill 1 octagon: 2 -7.62,1.143; 3 -5.08,-1.143; 4 -5.08,1.397; 5 -2.54,-1.397; 6 -2.54,1.143; 7 0,-1.143; 8 0,1.397; 9 2.54,-1.397; 10 2.54,1.143; 11 5.08,-1.143; 12 5.08,1.397; 13 7.62,-1.397; 14 7.62,1.143
FAB20B-3 = drill 1 octagon: A1 -1.27,11.43; A2 -1.27,8.89; A3 -1.27,6.35; A4 -1.27,3.81; A5 -1.27,1.27; A6 -1.27,-1.27; A7 -1.27,-3.81; A8 -1.27,-6.35; A9 -1.27,-8.89; A10 -1.27,-11.43; B1 1.27,11.43; B2 1.27,8.89; B3 1.27,6.35; B4 1.27,3.81; B5 1.27,1.27; B6 1.27,-1.27; B7 1.27,-3.81; B8 1.27,-6.35; B9 1.27,-8.89; B10 1.27,-11.43 | drill 2.8 pad 5.08: X1 0.965,17.06; X2 0.965,-17.06
BN50V = drill 1 pad 1.778: 1 0,0 | drill 1.5 pad 3.429: 2 3.442,3.442; 3 -3.442,3.442; 4 -3.442,-3.442; 5 3.442,-3.442

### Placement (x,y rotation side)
C1  29.21,99.06 90 top
C2  28.14,114.3 90 top
C11  65.53,90.17 180 top
C12  71.5,59.99 270 top
C13  60.96,60.96 180 top
C14  62.23,55.88 180 top
C15  90.68,90.17 0 top
C16  94.26,59.31 180 top
C17  84.33,60.4 90 top
C18  84.33,54.1 270 top
C19  116.33,90.17 180 top
C20  122.3,59.99 270 top
C21  111.76,60.96 180 top
C22  113.03,55.88 180 top
C23  141.48,90.17 0 top
C24  145.06,59.31 180 top
C25  135.13,60.4 90 top
C26  135.13,54.1 270 top
C27  167.13,90.17 180 top
C28  173.1,59.99 270 top
C29  162.56,60.96 180 top
C30  163.83,55.88 180 top
C31  192.28,90.17 0 top
C32  195.86,59.31 180 top
C33  185.93,60.4 90 top
C34  185.93,54.1 270 top
C35  217.93,90.17 180 top
C36  223.9,59.99 270 top
C37  213.36,60.96 180 top
C38  214.63,55.88 180 top
C39  243.08,90.17 0 top
C40  246.66,59.31 180 top
C41  236.73,60.4 90 top
C42  236.73,54.1 270 top
C43  268.73,90.17 180 top
C44  274.7,59.99 270 top
C45  264.16,60.96 180 top
C46  265.43,55.88 180 top
C47  293.88,90.17 0 top
C48  297.46,59.31 180 top
C49  287.53,60.4 90 top
C50  287.53,54.1 270 top
C51  319.53,90.17 180 top
C52  325.5,59.99 270 top
C53  314.96,60.96 180 top
C54  316.23,55.88 180 top
C55  344.68,90.17 0 top
C56  348.26,59.31 180 top
C57  338.33,60.4 90 top
C58  338.33,54.1 270 top
C59  370.33,90.17 180 top
C60  376.3,59.99 270 top
C61  365.76,60.96 180 top
C62  367.03,55.88 180 top
C63  395.48,90.17 0 top
C64  399.06,59.31 180 top
C65  389.13,60.4 90 top
C66  389.13,54.1 270 top
D1  16.51,96.52 180 bottom
D11  71.5,53.14 90 top
D12  95.14,55.19 180 top
D13  122.3,53.14 90 top
D14  145.94,55.19 180 top
D15  173.1,53.14 90 top
D16  196.74,55.19 180 top
D17  223.9,53.14 90 top
D18  247.54,55.19 180 top
D19  274.7,53.14 90 top
D20  298.34,55.19 180 top
D21  325.5,53.14 90 top
D22  349.14,55.19 180 top
D23  376.3,53.14 90 top
D24  399.94,55.19 180 top
DRILEGEND  [DRILEGEND]  not placed on the board
F1  36.83,100.84 0 bottom
F2  60.96,68.38 90 top
F3  95.25,68.38 270 top
F4  111.76,68.38 90 top
F5  146.05,68.38 270 top
F6  162.56,68.38 90 top
F7  196.85,68.38 270 top
F8  213.36,68.38 90 top
F9  247.65,68.38 270 top
F10  264.16,68.38 90 top
F11  298.45,68.38 270 top
F12  314.96,68.38 90 top
F13  349.25,68.38 270 top
F14  365.76,68.38 90 top
F15  400.05,68.38 270 top
IC1  35.56,96.52 270 bottom
K1  16.51,96.52 0 top
PM1  [PASSMARK]  not placed on the board
PM2  [PASSMARK]  not placed on the board
PM3  [PASSMARK]  not placed on the board
R1  39.37,92.71 90 bottom
R2  33.02,91.44 180 bottom
R3  26.67,91.44 90 bottom
X1  22.86,25.01 270 top
X2  48.56,64.35 0 top
X3  25.4,109.22 0 bottom
X4  34.29,87.63 180 top
X5  409.24,64.35 0 top
X6  305.3,13.97 180 top
X7  356.6,13.97 0 top
X8  305.3,114.3 180 top
X9  356.6,114.3 0 top
X11  77.77,64.35 0 top
X12  67.31,97.79 0 bottom
X13  67.31,55.88 270 bottom
X14  88.9,97.79 0 bottom
X15  88.9,55.88 270 bottom
X16  128.57,64.35 0 top
X17  118.11,97.79 0 bottom
X18  118.11,55.88 270 bottom
X19  139.7,97.79 0 bottom
X20  139.7,55.88 270 bottom
X21  179.37,64.35 0 top
X22  168.91,97.79 0 bottom
X23  168.91,55.88 270 bottom
X24  190.5,97.79 0 bottom
X25  190.5,55.88 270 bottom
X26  230.17,64.35 0 top
X27  219.71,97.79 0 bottom
X28  219.71,55.88 270 bottom
X29  241.3,97.79 0 bottom
X30  241.3,55.88 270 bottom
X31  280.97,64.35 0 top
X32  270.51,97.79 0 bottom
X33  270.51,55.88 270 bottom
X34  292.1,97.79 0 bottom
X35  292.1,55.88 270 bottom
X36  331.77,64.35 0 top
X37  321.31,97.79 0 bottom
X38  321.31,55.88 270 bottom
X39  342.9,97.79 0 bottom
X40  342.9,55.88 270 bottom
X41  382.57,64.35 0 top
X42  372.11,97.79 0 bottom
X43  372.11,55.88 270 bottom
X44  393.7,97.79 0 bottom
X45  393.7,55.88 270 bottom

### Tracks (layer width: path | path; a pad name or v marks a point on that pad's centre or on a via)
1-WIRE_1
  Bottom 0.254: X5.C17 413.41,63.08 416.31,65.98 416.31,112.27 414.1,114.48 375.07,114.48 370.32,109.73 359.9,109.73 357.87,111.76 357.87,114.43 X9.8
1-WIRE_2
  Bottom 0.254: X5.B21 410.5,51.66 413.41,51.66 416.31,48.77 416.31,16.51 414.02,14.22 372.09,14.22 368.54,17.78 359.01,17.78 X7.8
!PF
  Bottom 0.61: R1.1 39.37,52.07 43.58,47.87 X2.24 51.5,55.88 55.63,55.88 64.64,46.86 69.98,46.86 73.66,43.18 73.66,38.61 90.68,21.59 404.34,21.59 405.94,23.19 410,23.19 X5.C32
+3V3  (1 unrouted)
  Bottom 0.254: X5.B20 410.5,54.2 412.9,54.2 417.83,49.28 417.83,16 414.53,12.7 371.59,12.7 370.44,13.84 362.7,13.84 X7.11 | X5.C18 412.9,60.54 417.83,65.47 417.83,112.78 414.6,116 374.56,116 369.81,111.25 363.58,111.25 X9.11
+5V  (via drill 1)  (1 unrouted)
  Top 1.93: X5.C14 v422.27,70.7 | 411.75,70.7 X5.A14
  Bottom 1.93: X5.A14 X5.B14 X5.C14 | X8.4 312.92,117.34 315.98,120.4 420.62,120.4 423.55,117.47 423.55,71.97 v422.27,70.7 423.55,69.43 423.55,10.79 421.13,8.38 315.47,8.38 312.92,10.93 X6.4
+UB  (via drill 1)
  Top 0.813: v60.96,75.78 F2.2 | v365.76,75.78 F14.2 | v314.96,75.78 F12.2 | v264.16,75.78 F10.2 | v213.36,75.78 F8.2 | v162.56,75.78 F6.2 | v111.76,75.78 F4.2 | v95.25,75.78 F3.1 | v146.05,75.78 F5.1 | v196.85,75.78 F7.1 | v247.65,75.78 F9.1 | v298.45,75.78 F11.1 | v349.25,75.78 F13.1 | v400.05,75.78 F15.1
  Top 1.93: X6.1 295.14,11.43 83.82,11.43 62.48,32.77 62.48,45.85 57.15,51.18 57.15,54.61 48.56,63.2 48.56,73.27 X2.12
  Bottom 0.813: X2.4 40.12,98.67 | IC1.2 37.98,96.52 40.12,98.67 | 40.12,98.67 39.32,99.47 F1.1
  Bottom 1.93: X5.C12 X5.B12 X5.A12 v400.05,75.78 X41.B1 X41.A1 v365.76,75.78 v349.25,75.78 X36.B1 X36.A1 v314.96,75.78 v298.45,75.78 X31.B1 X31.A1 v264.16,75.78 v247.65,75.78 X26.B1 X26.A1 v213.36,75.78 v196.85,75.78 X21.B1 X21.A1 v162.56,75.78 v146.05,75.78 X16.B1 X16.A1 v111.76,75.78 v95.25,75.78 X11.B1 X11.A1 v60.96,75.78 58.4,78.34 X2.12 X2.8 X2.4 46.59,98.67 66.04,118.11 296.41,118.11 297.68,116.84 X8.1
-L  (via drill 0.5)
  Top 0.61: v48.26,82.55 46.99,83.82 40.64,83.82 36.96,87.5 X4.1 | v387.22,77.72 387.22,69 X41.B5 | v336.42,77.72 336.42,69 X36.B5 | v285.62,77.72 285.62,69 X31.B5 | v234.82,77.72 234.82,69 X26.B5 | v184.02,77.72 184.02,69 X21.B5 | v133.22,77.72 133.22,69 X16.B5 | v82.42,77.72 82.42,69 X11.B5
  Bottom 0.61: v48.26,82.55 50.42,80.39 59.31,80.39 61.98,77.72 v82.42,77.72 v133.22,77.72 v184.02,77.72 v234.82,77.72 v285.62,77.72 v336.42,77.72 v387.22,77.72 406.11,77.72 X5.A11
CANH_1
  Bottom 0.254: X5.B16 410.5,64.36 413.68,64.36 415.54,66.23 415.54,112.01 413.84,113.72 375.32,113.72 370.57,108.97 358.12,108.97 355.33,111.76 355.33,114.17 X9.6
CANH_2
  Bottom 0.254: X5.C22 413.68,50.38 415.54,48.51 415.54,16.76 413.77,14.99 372.35,14.99 368.79,18.54 357.49,18.54 X7.6
CANL_1
  Bottom 0.254: X5.C16 413.92,65.62 414.78,66.48 414.78,111.76 413.59,112.95 375.57,112.95 370.82,108.2 357.62,108.2 354.06,111.76 X9.5
CANL_2
  Bottom 0.254: X5.B22 410.5,49.12 413.92,49.12 414.78,48.26 414.78,17.02 413.51,15.75 372.6,15.75 369.05,19.3 355.58,19.3 352.79,16.51 352.79,13.84 X7.5
EXT_PNP_1
  Bottom 0.254: X5.C19 412.39,58 419.35,64.96 419.35,113.28 415.11,117.53 353.48,117.53 352.79,116.84 352.79,114.43 X9.3
EXT_PNP_2
  Top 0.254: X5.A20 407.96,54.2 414.93,54.2 419.35,49.78 419.35,15.49 415.04,11.18 353.17,11.18 X7.3
EXT_RESET_1
  Bottom 0.254: X5.A19 407.96,56.74 412.32,56.74 420.12,64.54 420.12,113.54 415.37,118.29 350.43,118.29 348.98,116.84 X9.2
EXT_RESET_2
  Top 0.254: X5.B19 410.5,56.74 414.86,56.74 420.12,51.49 420.12,15.24 415.29,10.41 351.27,10.41 350.25,11.43 350.25,13.84 X7.2
GND  (via drill 0.5, 1)
  Top 1.93: X2.10 X2.14
  Bottom 0.406: IC1.1 v36.96,98.07
  Bottom 0.813: IC1.4 33.52,95.57 v32.51,94.55 31.62,93.67 R2.1
  Bottom 1.93: X2.6 X2.10 | X2.14 53.67,73.24 X11.A2 X11.B2 v103.17,73.24 X16.A2 X16.B2 v153.97,73.24 X21.A2 X21.B2 v204.78,73.24 X26.A2 X26.B2 v255.57,73.24 X31.A2 X31.B2 v306.38,73.24 X36.A2 X36.B2 v357.18,73.24 X41.A2 X41.B2 X5.A13 X5.B13 X5.C13
  other vias: 103.17,79.59 153.97,79.59 204.77,79.59 255.57,79.59 306.37,79.59 357.17,79.59 418.13,58 88.9,79.59 67.31,79.59 118.11,79.59 139.7,79.59 190.5,79.59 168.91,79.59 219.71,79.59 241.3,79.59 270.51,79.59 292.1,79.59 321.31,79.59 342.9,79.59 372.11,79.59 393.7,79.59 78.11,101.23 128.91,101.23 179.71,101.23 230.5,101.23 281.31,101.23 332.11,101.23 382.9,101.23 419.4,55.46 419.4,60.54 342.9,83.4 372.11,83.4 393.7,83.4 321.31,83.4 292.1,83.4 270.51,83.4 241.3,83.4 219.71,83.4 190.5,83.4 168.91,83.4 139.7,83.4 118.11,83.4 88.9,83.4 67.31,83.4 382.9,94.35 332.11,94.35 281.31,94.35 230.5,94.35 179.71,94.35 128.91,94.35 78.11,94.35
  pour Bottom (isolate 0.305): 1.27,127.43 425.45,127.43 425.45,1.27 60.96,1.27 60.96,45.09 55.5,50.55 51.18,50.55 46.1,45.47 36.83,45.47 36.83,85.94 1.27,85.94
  pour Top (isolate 0.305): 1.27,127.43 425.45,127.43 425.45,1.27 60.96,1.27 60.96,45.09 55.5,50.55 51.18,50.55 46.1,45.47 36.83,45.47 36.83,85.94 1.27,85.94
L
  Bottom 1.93: X2.26 48.56,37.7 X2.28 35.67,37.7 28.05,30.09 X1.1
MESSSIG_1
  Top 0.813: C14.1 X13.3
  Bottom 0.61: X11.A4 72.39,64.05 72.39,58.42 69.85,55.88 X13.3
MESSSIG_2
  Top 0.813: C18.1 84.71,55.88 X15.3
  Bottom 0.61: X11.B4 83.82,63.38 83.82,57.15 85.09,55.88 X15.3
MESSSIG_3
  Top 0.813: C22.1 X18.3
  Bottom 0.61: X16.A4 123.19,64.05 123.19,58.42 120.65,55.88 X18.3
MESSSIG_4
  Top 0.813: C26.1 135.51,55.88 X20.3
  Bottom 0.61: X16.B4 134.62,63.38 134.62,57.15 135.89,55.88 X20.3
MESSSIG_5
  Top 0.813: C30.1 X23.3
  Bottom 0.61: X21.A4 173.99,64.05 173.99,58.42 171.45,55.88 X23.3
MESSSIG_6
  Top 0.813: C34.1 186.31,55.88 X25.3
  Bottom 0.61: X21.B4 185.42,63.38 185.42,57.15 186.69,55.88 X25.3
MESSSIG_7
  Top 0.813: C38.1 X28.3
  Bottom 0.61: X26.A4 224.79,64.05 224.79,58.42 222.25,55.88 X28.3
MESSSIG_8
  Top 0.813: C42.1 237.11,55.88 X30.3
  Bottom 0.61: X26.B4 236.22,63.38 236.22,57.15 237.49,55.88 X30.3
MESSSIG_9
  Top 0.813: C46.1 X33.3
  Bottom 0.61: X31.A4 275.59,64.05 275.59,58.42 273.05,55.88 X33.3
MESSSIG_10
  Top 0.813: C50.1 287.91,55.88 X35.3
  Bottom 0.61: X31.B4 287.02,63.38 287.02,57.15 288.29,55.88 X35.3
MESSSIG_11
  Top 0.813: C54.1 X38.3
  Bottom 0.61: X36.A4 326.39,64.05 326.39,58.42 323.85,55.88 X38.3
MESSSIG_12
  Top 0.813: C58.1 338.71,55.88 X40.3
  Bottom 0.61: X36.B4 337.82,63.38 337.82,57.15 339.09,55.88 X40.3
MESSSIG_13
  Top 0.813: C62.1 X43.3
  Bottom 0.61: X41.A4 377.19,64.05 377.19,58.42 374.65,55.88 X43.3
MESSSIG_14
  Top 0.813: C66.1 389.51,55.88 X45.3
  Bottom 0.61: X41.B4 388.62,63.38 388.62,57.15 389.89,55.88 X45.3
N
  Bottom 1.93: X2.30 39.61,32.62 31.99,25 X1.2
N$1
  Bottom 0.813: K1.1 12.83,90.04 R3.1
  Bottom 1.016: K1.1 10.16,93.98 12.7,96.52 D1.1
N$2
  Bottom 0.61: IC1.3 36.96,95.25 | 36.96,95.25 38.1,94.11 R1.2 | 36.96,95.25 34.42,92.71 R2.2
N$3
  Bottom 1.016: 22.86,93.98 20.32,96.52 D1.2 | K1.6 22.86,93.98 | 22.86,93.98 26.94,98.06 C1.+
N$4
  Bottom 0.813: IC1.5 32.57,97.47 27.94,92.84 R3.2
N$5
  Bottom 0.61: X3.6 21.29,101.91 K1.7
N$6
  Top 0.61: K1.10 15.24,105.41 19.91,110.08 X3.1
N$7
  Bottom 0.61: K1.12 19.05,109.22 21.23,109.22 X3.2
N$8
  Top 0.813: X3.4 C2.1
  Bottom 0.813: X3.4 28.78,110.64 34.15,105.27 34.29,105.13 34.34,105.08 F1.2
N$9
  Top 0.813: X13.4 64.7,58.62 C13.1 62.36,62.73 60.96,64.14 F2.1
N$10
  Top 0.813: F3.2 94.1,65.89 87.48,59.26 X15.4 84.71,58.62 C17.1
N$11
  Top 0.813: X18.4 115.5,58.62 C21.1 113.16,62.73 111.76,64.14 F4.1
N$12
  Top 0.813: X28.4 217.1,58.62 C37.1 214.76,62.73 213.36,64.14 F8.1
N$13
  Top 2: 10,-1 -1,-1 -1,10
N$14
  Top 2: 416.72,-1 427.72,-1 427.72,10
N$15
  Top 2: 34.56,56.03 34.56,45.03 23.56,45.03
N$16
  Top 2: 427.72,118.7 427.72,129.7 416.72,129.7
N$17
  Bottom 2: 10,-1 -1,-1 -1,10
N$18
  Bottom 2: 416.72,-1 427.72,-1 427.72,10
N$19
  Bottom 2: 23.56,45.03 34.56,45.03 34.56,56.03
N$20
  Bottom 2: 427.72,118.7 427.72,129.7 416.72,129.7
N$21
  Top 0.813: X23.4 166.3,58.62 C29.1 163.96,62.73 162.56,64.14 F6.1
N$22
  Top 0.813: X33.4 267.9,58.62 C45.1 265.56,62.73 264.16,64.14 F10.1
N$23
  Top 0.813: X38.4 318.7,58.62 C53.1 316.36,62.73 314.96,64.14 F12.1
N$24
  Top 0.813: X43.4 369.5,58.62 C61.1 367.16,62.73 365.76,64.14 F14.1
N$25
  Top 0.813: F5.2 144.9,65.89 138.28,59.26 X20.4 135.51,58.62 C25.1
N$26
  Top 0.813: F7.2 195.7,65.89 189.08,59.26 X25.4 186.31,58.62 C33.1
N$27
  Top 0.813: F9.2 246.5,65.89 239.88,59.26 X30.4 237.11,58.62 C41.1
N$28
  Top 0.813: F15.2 398.9,65.89 392.28,59.26 X45.4 389.51,58.62 C65.1
N$29
  Top 0.813: F13.2 348.1,65.89 341.48,59.26 X40.4 338.71,58.62 C57.1
N$30
  Top 0.813: F11.2 297.3,65.89 290.68,59.26 X35.4 287.91,58.62 C49.1
N$45
  Bottom 2: 10,129.7 -1,129.7 -1,118.7
N$46
  Top 2: 10,129.7 -1,129.7 -1,118.7
N$47
  Bottom 2: 10,45.03 -1,45.03 -1,34.03
N$48
  Top 2: 10,45.03 -1,45.03 -1,34.03
N$49
  Top 2: 23.56,83.67 34.56,83.67 34.56,72.67
N$50
  Bottom 2: 34.56,72.67 34.56,83.67 23.56,83.67
N$51
  Top 2: 10,83.67 -1,83.67 -1,94.67
N$52
  Bottom 2: -1,94.67 -1,83.67 10,83.67
OEFFNER_1
  Bottom 0.406: X11.A9 77.78,54.19 77.78,51.61 74.93,48.77 74.93,39.37 91.44,22.86 403.81,22.86 405.93,24.98 X5.A32
  Bottom 0.61: X13.2 65.89,52.48 68.45,49.91 70.96,49.91 X11.A9
OEFFNER_2
  Bottom 0.406: X15.2 87.48,52.48 93.98,45.97 93.98,39.37 109.22,24.13 403.3,24.13 405.41,26.24 407.96,26.24 X5.B31
  Bottom 0.61: X11.B9 81.37,53.14 X15.2
OEFFNER_3
  Bottom 0.406: X16.A9 128.57,54.19 128.57,51.61 125.73,48.77 125.73,39.37 139.7,25.4 402.79,25.4 406.17,28.78 410.5,28.78 X5.C30
  Bottom 0.61: X18.2 116.69,52.48 119.25,49.91 121.76,49.91 X16.A9
OEFFNER_4
  Bottom 0.406: X20.2 138.28,52.48 144.78,45.97 144.78,39.37 157.48,26.67 402.29,26.67 405.68,30.06 X5.A30
  Bottom 0.61: X16.B9 132.17,53.14 X20.2
OEFFNER_5
  Bottom 0.406: X21.A9 179.38,54.19 179.38,51.61 176.53,48.77 176.53,39.37 187.96,27.94 401.78,27.94 405.15,31.32 407.96,31.32 X5.B29
  Bottom 0.61: X23.2 167.49,52.48 170.05,49.91 172.56,49.91 X21.A9
OEFFNER_6
  Bottom 0.406: X25.2 189.08,52.48 195.58,45.97 195.58,39.37 205.74,29.21 401.27,29.21 405.92,33.86 410.5,33.86 X5.C28
  Bottom 0.61: X21.B9 182.97,53.14 X25.2
OEFFNER_7
  Bottom 0.406: X26.A9 230.18,54.19 230.18,51.61 227.33,48.77 227.33,39.37 236.22,30.48 400.76,30.48 405.42,35.14 X5.A28
  Bottom 0.61: X28.2 218.29,52.48 220.85,49.91 223.36,49.91 X26.A9
OEFFNER_8
  Bottom 0.406: X30.2 239.88,52.48 246.38,45.97 246.38,39.37 254,31.75 400.25,31.75 404.9,36.4 407.96,36.4 X5.B27
  Bottom 0.61: X26.B9 233.77,53.14 X30.2
OEFFNER_9
  Bottom 0.406: X31.A9 280.98,54.19 280.98,51.61 278.13,48.77 278.13,39.37 284.48,33.02 399.75,33.02 405.66,38.94 410.5,38.94 X5.C26
  Bottom 0.61: X33.2 269.09,52.48 271.65,49.91 274.16,49.91 X31.A9
OEFFNER_10
  Bottom 0.406: X35.2 290.68,52.48 297.18,45.97 297.18,39.37 302.26,34.29 399.24,34.29 405.17,40.22 X5.A26
  Bottom 0.61: X31.B9 284.57,53.14 X35.2
OEFFNER_11
  Bottom 0.406: X36.A9 331.77,54.19 331.77,51.61 328.93,48.77 328.93,39.37 332.74,35.56 398.73,35.56 404.65,41.48 407.96,41.48 X5.B25
  Bottom 0.61: X38.2 319.89,52.48 322.45,49.91 324.96,49.91 X36.A9
OEFFNER_12
  Bottom 0.406: X40.2 341.48,52.48 347.98,45.97 347.98,39.37 350.52,36.83 398.22,36.83 405.41,44.02 410.5,44.02 X5.C24
  Bottom 0.61: X36.B9 335.37,53.14 X40.2
OEFFNER_13
  Bottom 0.406: X41.A9 382.57,54.19 382.57,51.61 379.73,48.77 379.73,39.37 381,38.1 397.71,38.1 404.91,45.3 X5.A24
  Bottom 0.61: X43.2 370.69,52.48 373.25,49.91 375.76,49.91 X41.A9
OEFFNER_14
  Bottom 0.406: X5.B23 407.96,46.56 398.22,46.56 392.28,52.5 X45.2
  Bottom 0.61: X41.B9 386.17,53.14 X45.2
PE  (via drill 2.8 pad 5.08)
  Bottom 1.93: X2.32 35.87,19.93 X1.3
  other vias: 17.78,3.1 48.26,3.1
  pour Bottom (isolate 0.305, no thermals): 1.27,42.76 30.06,42.76 25.4,38.1 17.78,38.1 13.97,34.29 13.97,24.13 17.35,20.75 35.51,20.75 43.13,28.37 45.01,28.37 49.25,24.13 55.88,24.13 55.88,1.27 1.27,1.27
  pour Top (isolate 0.305, no thermals): 1.27,42.76 30.06,42.76 25.4,38.1 17.78,38.1 13.97,34.29 13.97,24.13 17.35,20.75 35.51,20.75 43.13,28.37 45.01,28.37 49.25,24.13 55.88,24.13 55.88,1.27 1.27,1.27
RESET_1
  Top 0.254: X11.A3 74.93,72.28 74.93,102.87 82.55,110.49 402.77,110.49 407.85,105.41 410.1,105.41 X5.C1
  Top 0.813: X13.8 70.1,57.25 | 70.1,57.25 70.16,57.25 C12.2 | D11.2 71.5,55.85 70.1,57.25
  Bottom 0.61: X11.A3 71.12,65.31 71.12,59.64 X13.8
RESET_2
  Top 0.254: X5.A1 406.7,105.79 402.51,109.98 89.28,109.98 82.17,102.87 82.17,79.63 80.64,78.11 80.64,72.3 X11.B3
  Top 0.813: X15.8 90.8,57.25 | 90.8,57.25 C16.2 | D12.2 90.8,57.25
  Bottom 0.61: X11.B3 85.09,64.66 85.09,58.42 86.26,57.25 X15.8
RESET_3
  Top 0.254: X16.A3 125.73,72.28 125.73,102.87 132.33,109.47 402.26,109.47 405.44,106.3 405.44,103.25 406.25,102.44 410.53,102.44 X5.C2
  Top 0.813: X18.8 120.96,57.25 | 120.96,57.25 C20.2 | D13.2 122.3,55.91 120.96,57.25
  Bottom 0.61: X16.A3 121.92,65.31 121.92,59.64 X18.8
RESET_4
  Top 0.254: X5.A2 404.93,102.96 404.93,106.05 402.01,108.97 139.06,108.97 132.97,102.87 132.97,79.63 131.44,78.11 131.44,72.3 X16.B3
  Top 0.813: X20.8 141.6,57.25 | 141.6,57.25 C24.2 | D14.2 141.6,57.25
  Bottom 0.61: X16.B3 135.89,64.66 135.89,58.42 137.06,57.25 X20.8
RESET_5
  Top 0.254: X21.A3 176.53,72.28 176.53,102.87 182.12,108.46 401.75,108.46 404.42,105.79 404.42,101.73 406.25,99.9 410.53,99.9 X5.C3
  Top 0.813: X23.8 171.76,57.25 | 171.76,57.25 C28.2 | D15.2 173.1,55.91 171.76,57.25
  Bottom 0.61: X21.A3 172.72,65.31 172.72,59.64 X23.8
RESET_6
  Top 0.254: X5.A3 403.91,101.43 403.91,105.54 401.5,107.95 188.85,107.95 183.77,102.87 183.77,79.63 182.25,78.11 182.25,72.3 X21.B3
  Top 0.813: X25.8 192.4,57.25 | 192.4,57.25 C32.2 | D16.2 192.4,57.25
  Bottom 0.61: X21.B3 186.69,64.66 186.69,58.42 187.86,57.25 X25.8
RESET_7
  Top 0.254: X26.A3 227.33,72.28 227.33,102.87 231.9,107.44 401.24,107.44 403.4,105.28 403.4,100.2 406.25,97.36 410.53,97.36 X5.C4
  Top 0.813: X28.8 222.56,57.25 | 222.56,57.25 C36.2 | D17.2 223.9,55.91 222.56,57.25
  Bottom 0.61: X26.A3 223.52,65.31 223.52,59.64 X28.8
RESET_8
  Top 0.254: X5.A4 402.89,99.91 402.89,105.03 400.99,106.93 238.63,106.93 234.57,102.87 234.57,79.63 233.04,78.11 233.04,72.3 X26.B3
  Top 0.813: X30.8 243.2,57.25 | 243.2,57.25 C40.2 | D18.2 243.2,57.25
  Bottom 0.61: X26.B3 237.49,64.66 237.49,58.42 238.66,57.25 X30.8
RESET_9
  Top 0.254: X31.A3 278.13,72.28 278.13,102.87 281.69,106.43 400.74,106.43 402.39,104.78 402.39,98.68 406.25,94.82 407.99,94.82 X5.B5
  Top 0.813: X33.8 273.3,57.25 | 273.3,57.25 273.36,57.25 C44.2 | D19.2 274.7,55.85 273.3,57.25
  Bottom 0.61: X31.A3 274.32,65.31 274.32,59.64 X33.8
RESET_10
  Top 0.254: X5.B6 407.99,92.28 406.25,92.28 401.88,96.65 401.88,104.52 400.48,105.92 288.42,105.92 285.37,102.87 285.37,79.63 283.85,78.11 283.85,72.3 X31.B3
  Top 0.813: X35.8 294,57.25 | 294,57.25 C48.2 | D20.2 294,57.25
  Bottom 0.61: X31.B3 288.29,64.66 288.29,58.42 289.46,57.25 X35.8
RESET_11
  Top 0.254: X36.A3 328.93,72.28 328.93,102.87 331.47,105.41 400.23,105.41 401.37,104.27 401.37,94.61 406.25,89.74 407.99,89.74 X5.B7
  Top 0.813: X38.8 324.1,57.25 | 324.1,57.25 324.16,57.25 C52.2 | D21.2 325.5,55.85 324.1,57.25
  Bottom 0.61: X36.A3 325.12,65.31 325.12,59.64 X38.8
RESET_12
  Top 0.254: X5.B8 407.99,87.2 406.25,87.2 400.86,92.58 400.86,104.01 399.97,104.9 338.2,104.9 336.17,102.87 336.17,79.63 334.64,78.11 334.64,72.3 X36.B3
  Top 0.813: X40.8 344.8,57.25 | 344.8,57.25 C56.2 | D22.2 344.8,57.25
  Bottom 0.61: X36.B3 339.09,64.66 339.09,58.42 340.26,57.25 X40.8
RESET_13
  Top 0.254: X5.B9 407.99,84.66 406.25,84.66 400.36,90.55 400.36,103.76 399.72,104.39 381.25,104.39 379.73,102.87 379.73,72.28 X41.A3
  Top 0.813: X43.8 374.96,57.25 | 374.96,57.25 C60.2 | D23.2 376.3,55.91 374.96,57.25
  Bottom 0.61: X41.A3 375.92,65.31 375.92,59.64 X43.8
RESET_14
  Top 0.254: X5.B10 407.99,82.12 406.25,82.12 399.85,88.52 399.85,103.5 399.47,103.89 387.99,103.89 386.97,102.87 386.97,79.63 385.44,78.11 385.44,72.3 X41.B3
  Top 0.813: X45.8 395.6,57.25 | 395.6,57.25 C64.2 | D24.2 397.66,55.35 397.5,55.35 395.6,57.25
  Bottom 0.61: X41.B3 389.89,64.66 389.89,58.42 391.06,57.25 X45.8
SCHLIESSER_1
  Bottom 0.61: X11.A10 71.84,48.26 68.02,48.26 X13.1
SCHLIESSER_2
  Bottom 0.61: X11.B10 81.57,50.39 X15.1
SCHLIESSER_3
  Bottom 0.61: X16.A10 122.64,48.26 118.82,48.26 X18.1
SCHLIESSER_4
  Bottom 0.61: X16.B10 132.37,50.39 X20.1
SCHLIESSER_5
  Bottom 0.61: X21.A10 173.44,48.26 169.62,48.26 X23.1
SCHLIESSER_6
  Bottom 0.61: X21.B10 183.17,50.39 X25.1
SCHLIESSER_7
  Bottom 0.61: X26.A10 224.25,48.26 220.42,48.26 X28.1
SCHLIESSER_8
  Bottom 0.61: X26.B10 233.97,50.39 X30.1
SCHLIESSER_9
  Bottom 0.61: X31.A10 275.05,48.26 271.22,48.26 X33.1
SCHLIESSER_10
  Bottom 0.61: X31.B10 284.77,50.39 X35.1
SCHLIESSER_11
  Bottom 0.61: X36.A10 325.85,48.26 322.02,48.26 X38.1
SCHLIESSER_12
  Bottom 0.61: X36.B10 335.57,50.39 X40.1
SCHLIESSER_13
  Bottom 0.61: X41.A10 376.64,48.26 372.82,48.26 X43.1
SCHLIESSER_14
  Bottom 0.61: X41.B10 386.37,50.39 X45.1
SCL_1
  Bottom 0.254: X5.B18 410.5,59.28 412.66,59.28 418.59,65.21 418.59,113.03 414.86,116.76 374.3,116.76 370.44,112.9 X9.13
SCL_2
  Bottom 0.254: X5.C20 412.66,55.46 418.59,49.53 418.59,15.75 414.78,11.94 371.33,11.94 370.7,12.57 X7.13
SDA_1
  Bottom 0.254: X5.B17 410.5,61.82 413.17,61.82 417.07,65.72 417.07,112.52 414.35,115.24 374.81,115.24 370.06,110.49 361.68,110.49 360.41,111.76 360.41,114.17 X9.10
SDA_2
  Bottom 0.254: X5.C21 413.17,52.92 417.07,49.02 417.07,16.26 414.27,13.46 371.84,13.46 368.28,17.02 361.05,17.02 X7.10
SONDE_1
  Top 0.813: C11.1 67.31,90.17
  Top 1.016: X12.1 67.31,90.17 67.31,88.9 72.39,83.82 72.39,67.19 X11.A6
  Bottom 0.254: X12.1 67.31,88.9 71.12,85.09 402.48,85.09 X5.A10
SONDE_2
  Top 0.813: C15.1 88.9,90.17
  Top 1.016: X14.1 88.9,90.17 88.9,88.9 83.82,83.82 83.82,67.86 X11.B6
  Bottom 0.254: X14.1 88.9,88.9 92.2,85.6 402.77,85.6 406.25,82.12 410.53,82.12 X5.C10
SONDE_3
  Top 0.813: C19.1 118.11,90.17
  Top 1.016: X17.1 118.11,90.17 118.11,88.9 123.19,83.82 123.19,67.19 X16.A6
  Bottom 0.254: X17.1 118.11,88.9 120.9,86.11 404,86.11 X5.A9
SONDE_4
  Top 0.813: C23.1 139.7,90.17
  Top 1.016: X19.1 139.7,90.17 139.7,88.9 134.62,83.82 134.62,67.86 X16.B6
  Bottom 0.254: X19.1 139.7,88.9 141.99,86.61 404.29,86.61 406.25,84.66 410.53,84.66 X5.C9
SONDE_5
  Top 0.813: C27.1 168.91,90.17
  Top 1.016: X22.1 168.91,90.17 168.91,88.9 173.99,83.82 173.99,67.19 X21.A6
  Bottom 0.254: X22.1 168.91,88.9 170.69,87.12 405.52,87.12 X5.A8
SONDE_6
  Top 0.813: 190.5,88.9 190.5,90.17 C31.1
  Top 1.016: X24.1 190.5,90.17 | 190.5,88.9 185.42,83.82 185.42,67.86 X21.B6
  Bottom 0.254: X24.1 190.5,88.9 191.77,87.63 405.82,87.63 406.25,87.2 410.53,87.2 X5.C8
SONDE_7
  Top 0.813: C35.1 219.71,90.17
  Top 1.016: X27.1 219.71,90.17 219.71,88.9 224.79,83.82 224.79,67.19 X26.A6
  Bottom 0.254: X27.1 219.71,88.9 220.47,88.14 406.36,88.14 X5.A7
SONDE_8
  Top 0.813: 241.3,88.9 241.3,90.17 C39.1
  Top 1.016: X29.1 241.3,90.17 | 241.3,88.9 236.22,83.82 236.22,67.86 X26.B6
  Bottom 0.254: X29.1 241.3,88.9 241.55,88.65 405.15,88.65 406.25,89.74 410.53,89.74 X5.C7
SONDE_9
  Top 0.813: C43.1 270.51,90.17
  Top 1.016: X32.1 270.51,90.17 270.51,88.9 275.59,83.82 275.59,67.19 X31.A6
  Bottom 0.254: X32.1 270.51,90.17 271.53,89.15 404.84,89.15 X5.A6
SONDE_10
  Top 0.813: C47.1 292.1,90.17
  Top 1.016: X34.1 292.1,90.17 292.1,88.9 287.02,83.82 287.02,67.86 X31.B6
  Bottom 0.254: X34.1 292.1,90.17 292.61,89.66 403.63,89.66 406.25,92.28 410.53,92.28 X5.C6
SONDE_11
  Top 0.813: C51.1 321.31,90.17
  Top 1.016: X37.1 321.31,90.17 321.31,88.9 326.39,83.82 326.39,67.19 X36.A6
  Bottom 0.254: X37.1 321.31,91.44 322.58,90.17 403.31,90.17 X5.A5
SONDE_12
  Top 0.813: C55.1 342.9,90.17
  Top 1.016: X39.1 342.9,90.17 342.9,88.9 337.82,83.82 337.82,67.86 X36.B6
  Bottom 0.254: X39.1 342.9,91.44 343.66,90.68 402.11,90.68 406.25,94.82 410.53,94.82 X5.C5
SONDE_13
  Top 0.813: C59.1 372.11,90.17
  Top 1.016: X42.1 372.11,90.17 372.11,88.9 377.19,83.82 377.19,67.19 X41.A6
  Bottom 0.254: X42.1 372.11,91.44 372.36,91.19 400.07,91.19 406.25,97.36 407.99,97.36 X5.B4
SONDE_14
  Top 0.813: C63.1 393.7,90.17
  Top 1.016: X44.1 393.7,90.17 393.7,88.9 388.62,83.82 388.62,67.86 X41.B6
  Bottom 0.254: X5.B3 407.99,99.9 406.25,99.9 404.14,97.79 X44.1
WECHSLER_1
  Top 0.406: X5.B32 407.96,23.7 404.65,23.7 403.81,22.86 91.44,22.86 74.93,39.37 74.93,56.42 X11.A8
  Bottom 0.61: X11.A8 70.27,51.77 X13.6
WECHSLER_2
  Top 0.406: X5.C31 410.5,26.24 405.41,26.24 403.3,24.13 109.22,24.13 93.98,39.37 93.98,48.11 X15.6
  Bottom 0.61: X11.B8 82.56,54.48 88.27,54.48 90.32,52.43 X15.6
WECHSLER_3
  Top 0.406: X16.A8 125.73,56.42 125.73,39.37 139.7,25.4 402.79,25.4 404.91,27.52 X5.A31
  Bottom 0.61: X16.A8 121.07,51.77 X18.6
WECHSLER_4
  Top 0.406: X5.B30 407.96,28.78 404.39,28.78 402.29,26.67 157.48,26.67 144.78,39.37 144.78,48.11 X20.6
  Bottom 0.61: X16.B8 133.36,54.48 139.06,54.48 141.12,52.43 X20.6
WECHSLER_5
  Top 0.406: X21.A8 176.53,56.42 176.53,39.37 187.96,27.94 401.78,27.94 405.15,31.32 410.5,31.32 X5.C29
  Bottom 0.61: X21.A8 171.87,51.77 X23.6
WECHSLER_6
  Top 0.406: X5.A29 404.66,32.6 401.27,29.21 205.74,29.21 195.58,39.37 195.58,48.11 X25.6
  Bottom 0.61: X21.B8 184.16,54.48 189.87,54.48 191.92,52.43 X25.6
WECHSLER_7
  Top 0.406: X26.A8 227.33,56.42 227.33,39.37 236.22,30.48 400.76,30.48 404.14,33.86 407.96,33.86 X5.B28
  Bottom 0.61: X26.A8 222.67,51.77 X28.6
WECHSLER_8
  Top 0.406: X5.C27 410.5,36.4 404.9,36.4 400.25,31.75 254,31.75 246.38,39.37 246.38,48.11 X30.6
  Bottom 0.61: X26.B8 234.96,54.48 240.66,54.48 242.72,52.43 X30.6
WECHSLER_9
  Top 0.406: X31.A8 278.13,56.42 278.13,39.37 284.48,33.02 399.75,33.02 404.4,37.68 X5.A27
  Bottom 0.61: X31.A8 273.47,51.77 X33.6
WECHSLER_10
  Top 0.406: X5.B26 407.96,38.94 403.88,38.94 399.24,34.29 302.26,34.29 297.18,39.37 297.18,48.11 X35.6
  Bottom 0.61: X31.B8 285.76,54.48 291.46,54.48 293.52,52.43 X35.6
WECHSLER_11
  Top 0.406: X36.A8 328.93,56.42 328.93,39.37 332.74,35.56 398.73,35.56 404.65,41.48 410.5,41.48 X5.C25
  Bottom 0.61: X36.A8 324.27,51.77 X38.6
WECHSLER_12
  Top 0.406: X5.A25 404.15,42.76 398.22,36.83 350.52,36.83 347.98,39.37 347.98,48.11 X40.6
  Bottom 0.61: X36.B8 336.56,54.48 342.26,54.48 344.32,52.43 X40.6
WECHSLER_13
  Top 0.406: X5.B24 407.96,44.02 403.63,44.02 397.71,38.1 381,38.1 379.73,39.37 379.73,56.42 X41.A8
  Bottom 0.61: X41.A8 375.07,51.77 X43.6
WECHSLER_14
  Top 0.406: X5.A23 405.42,46.56 398.22,46.56 395.12,49.66 X45.6
  Bottom 0.61: X41.B8 387.36,54.48 393.06,54.48 395.12,52.43 X45.6

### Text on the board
Top: Absorberüberwachung Backplane 2015-09-20 MH | Rev. 2.4 | Top
Bottom: Bottom
tPlace: X8 | X9 | C2 | 1 | C1 | K1 | X4 | 1 | C11 | C15 | C19 | C23 | C27 | C31 | C35 | C39 | C43 | C47 | C51 | C55 | C59 | C63 | F2 | F3 | F4 | F5 | F6 | F7 | F8 | F9 | F10 | F11 | F12 | F13 | F14 | F15 | C17 | C25 | C35 | C41 | C49 | C57 | C65 | C12 | C20 | C28 | C36 | C44 | C52 | C60 | C13 | C21 | C29 | C37 | C45 | C53 | C61 | C16 | C24 | C32 | C40 | C48 | C56 | C64 | C14 | C22 | C30 | C38 | C46 | C54 | C62 | D12 | D14 | D16 | D18 | D20 | D22 | D24 | 1 | 1 | 1 | 1 | 1 | 1 | 1 | 1 | 1 | 1 | 1 | 1 | 1 | 1 | D11 | D13 | D15 | D17 | D19 | D21 | D23 | C18 | C26 | C34 | C42 | C50 | C58 | C66 | X11 | X16 | X21 | X26 | X31 | X36 | X41 | 5 | L | 9 | 4 | Reset | 8 | +Ub | 3 | N | datacrumbs | GND | 7 | Messsignal | 2 | Wechsler | Öffner | 6 | PE | 1 | Schließer | X6 | X7 | X1 | X2 | X5
bPlace: X3 | 1 | b1a | X12 | X14 | X17 | X19 | X22 | X24 | X27 | X29 | X32 | X34 | X37 | X39 | X42 | X44 | F1 | D1 | R3 | R2 | R1 | IC1 | 1 | 1a | 1a | 1a | 1a | 1a | 1a | 1a | X13 | X15 | X18 | X20 | X23 | X25 | X28 | X30 | X33 | X35 | X38 | X40 | X43 | X45 | 1 | 5 | L | 9 | 4 | +Ub | 8 | Reset | 3 | N | datacrumbs | Messsignal | 7 | GND | 2 | Öffner | Wechsler | 6 | PE | 1 | Schließer | 1
DrillLegend: LAYER-STACK
DrillLegend_01-16: 01-16
DrillLegend_01-20: 01-20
